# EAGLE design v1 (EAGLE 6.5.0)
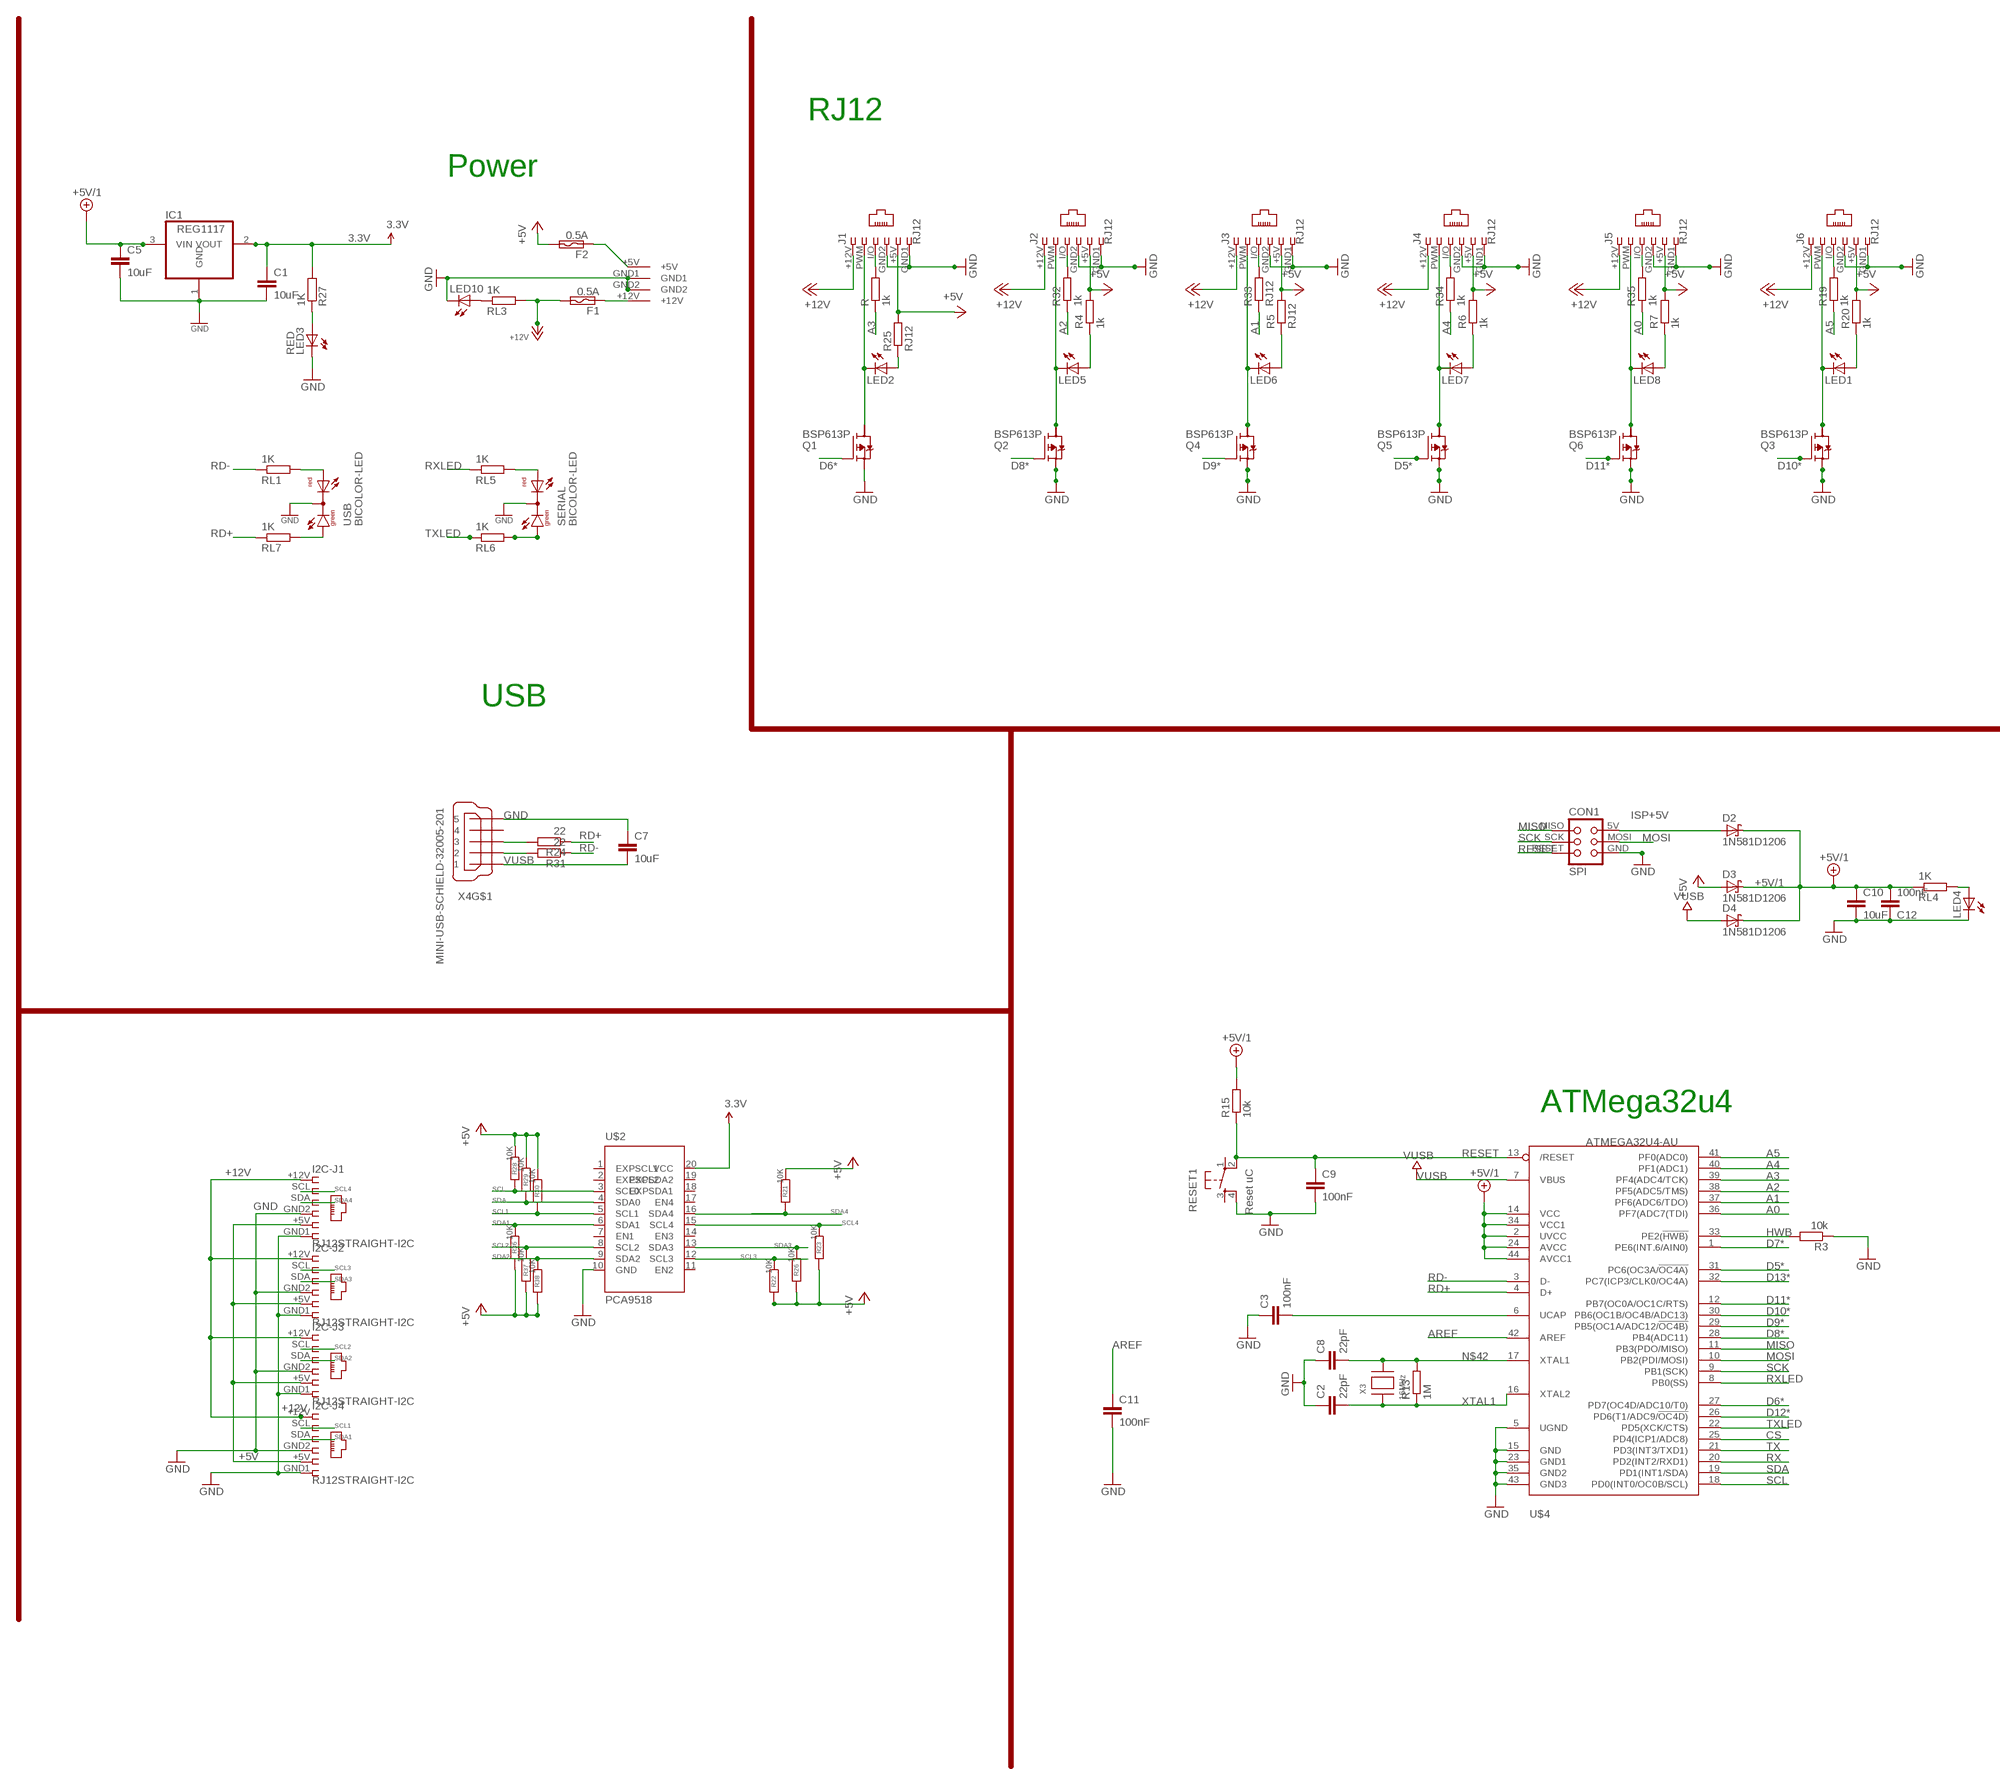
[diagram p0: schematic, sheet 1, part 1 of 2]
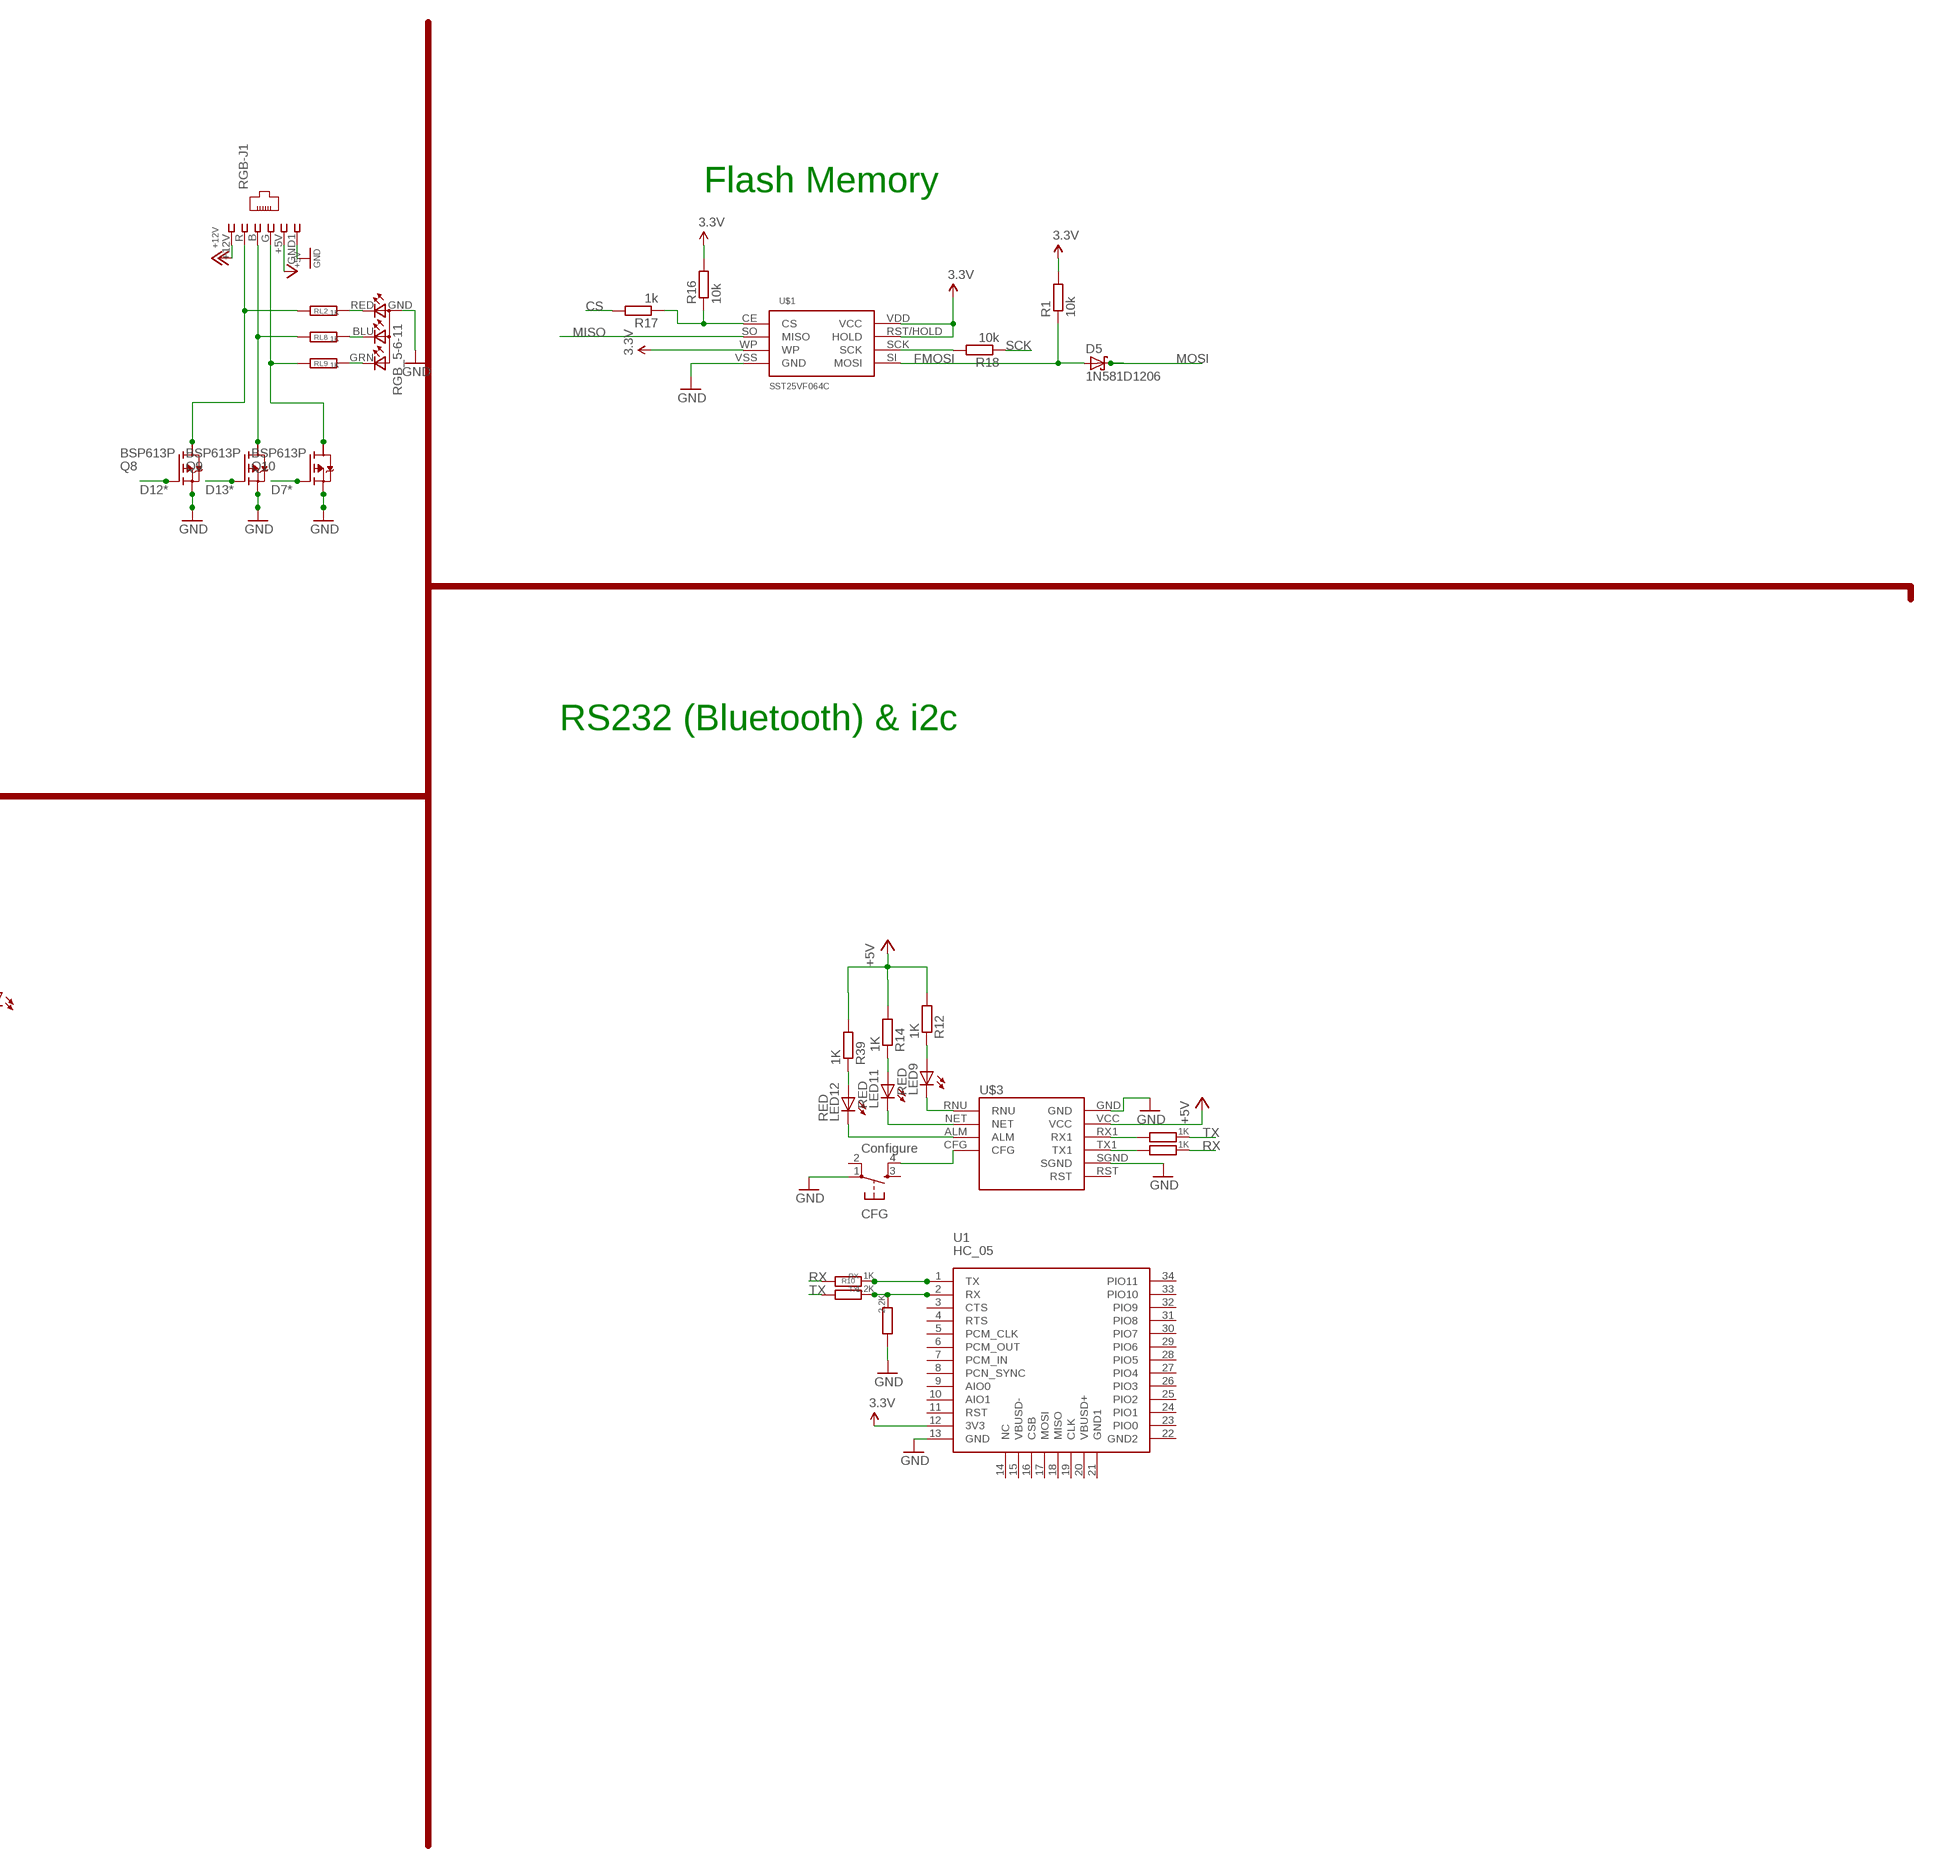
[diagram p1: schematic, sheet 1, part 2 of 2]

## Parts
C1  10uF  C-EUC1206  [C1206]
C2  22pF  C-EUC1206  [C1206]
C3  100nF  C-EUC1206  [C1206]
C5  10uF  C-EUC1206  [C1206]
C7  10uF  C-EUC1206  [C1206]
C8  22pF  C-EUC1206  [C1206]
C9  100nF  C-EUC1206  [C1206]
C10  10uF  C-EUC1206  [C1206]
C11  100nF  C-EUC1206  [C1206]
C12  100nF  C-EUC1206  [C1206]
CFG  Configure  TAC_SWITCHSMD  [TACTILE_SWITCH_SMD]
CON1  SPI  TINYISPT  [TC2030-MCP-NL]
D2  1N581D1206  [LED-1206]
D3  1N581D1206  [LED-1206]
D4  1N581D1206  [LED-1206]
D5  1N581D1206  [LED-1206]
F1  0.5A  POLYSWITCHSMD1812  [C1812]
F2  0.5A  POLYSWITCHSMD1812  [C1812]
I2C-J1  RJ12STRAIGHT-I2C  [RJ12-STRAIGHT-I2C]
I2C-J2  RJ12STRAIGHT-I2C  [RJ12-STRAIGHT-I2C]
I2C-J3  RJ12STRAIGHT-I2C  [RJ12-STRAIGHT-I2C]
I2C-J4  RJ12STRAIGHT-I2C  [RJ12-STRAIGHT-I2C]
IC1  REG1117  [SOT223]
J1  RJ12  RJ12STRAIGHT  [RJ12-STRAIGHT]
J2  RJ12  RJ12STRAIGHT  [RJ12-STRAIGHT]
J3  RJ12  RJ12STRAIGHT  [RJ12-STRAIGHT]
J4  RJ12  RJ12STRAIGHT  [RJ12-STRAIGHT]
J5  RJ12  RJ12STRAIGHT  [RJ12-STRAIGHT]
J6  RJ12  RJ12STRAIGHT  [RJ12-STRAIGHT]
LED1  Blue  LED3MM  [LED3MM]
LED2  Blue  LED3MM  [LED3MM]
LED3  RED  LEDCHIP-LED0805  [CHIP-LED0805]
LED4  RED  LED3MM  [LED3MM]
LED5  Blue  LED3MM  [LED3MM]
LED6  Blue  LED3MM  [LED3MM]
LED7  BLue  LED3MM  [LED3MM]
LED8  Blue  LED3MM  [LED3MM]
LED9  RED  LEDCHIP-LED0805  [CHIP-LED0805]
LED10  RED  LED3MM  [LED3MM]
LED11  RED  LEDCHIP-LED0805  [CHIP-LED0805]
LED12  RED  LEDCHIP-LED0805  [CHIP-LED0805]
Q1  BSP613P  [PG-SOT-223]
Q2  BSP613P  [PG-SOT-223]
Q3  BSP613P  [PG-SOT-223]
Q4  BSP613P  [PG-SOT-223]
Q5  BSP613P  [PG-SOT-223]
Q6  BSP613P  [PG-SOT-223]
Q8  BSP613P  [PG-SOT-223]
Q9  BSP613P  [PG-SOT-223]
Q10  BSP613P  [PG-SOT-223]
R  1k  R-EU_R0805  [R0805]
R1  10k  R-EU_R1206  [R1206]
R2  2.2K  R-EU_R0805  [R0805]
R3  10k  R-EU_M0805  [M0805]
R4  1k  R-EU_R0805  [R0805]
R5  RJ12  R-EU_R0805  [R0805]
R6  1k  R-EU_R0805  [R0805]
R7  1k  R-EU_R0805  [R0805]
R8  1K  R-EU_R0805  [R0805]
R9  1.2K  R-EU_R0805  [R0805]
R10  1K  R-EU_R0805  [R0805]
R11  1K  R-EU_R0805  [R0805]
R12  1K  R-EU_R0805  [R0805]
R13  1M  R-EU_R1206  [R1206]
R14  1K  R-EU_R0805  [R0805]
R15  10k  R-EU_M0805  [M0805]
R16  10k  R-EU_R1206  [R1206]
R17  1k  R-EU_R0805  [R0805]
R18  10k  R-EU_R1206  [R1206]
R19  1k  R-EU_R0805  [R0805]
R20  1k  R-EU_R0805  [R0805]
R21  10K  R-EU_M0805  [M0805]
R22  10K  R-EU_M0805  [M0805]
R23  10K  R-EU_M0805  [M0805]
R24  22  R-EU_M1206  [M1206]
R25  RJ12  R-EU_R0805  [R0805]
R26  10K  R-EU_M0805  [M0805]
R27  1K  R-EU_R0805  [R0805]
R28  10K  R-EU_M0805  [M0805]
R29  10K  R-EU_M0805  [M0805]
R30  10K  R-EU_M0805  [M0805]
R31  22  R-EU_M1206  [M1206]
R32  1k  R-EU_R0805  [R0805]
R33  RJ12  R-EU_R0805  [R0805]
R34  1k  R-EU_R0805  [R0805]
R35  1k  R-EU_R0805  [R0805]
R36  10K  R-EU_M0805  [M0805]
R37  10K  R-EU_M0805  [M0805]
R38  10K  R-EU_M0805  [M0805]
R39  1K  R-EU_R0805  [R0805]
RESET1  Reset uC  TAC_SWITCHSMD  [TACTILE_SWITCH_SMD]
RGB-J1  RJ12  RJ12STRAIGHT-RGB  [RJ12-STRAIGHT-RGB]
RGB_5-6-11  TOPLED-3  [LED-TRICOLOR-THROUGHHOLE]
RL1  1K  R-EU_R0805  [R0805]
RL2  1K  R-EU_M0805  [M0805]
RL3  1K  R-EU_R0805  [R0805]
RL4  1K  R-EU_R0805  [R0805]
RL5  1K  R-EU_R0805  [R0805]
RL6  1K  R-EU_R0805  [R0805]
RL7  1K  R-EU_R0805  [R0805]
RL8  1K  R-EU_M0805  [M0805]
RL9  1K  R-EU_M0805  [M0805]
SERIAL  BICOLOR-LED  [BICOLOR-3MM]
U1  HC_05  [BLUETOOTH_SMD]
U$1  SST25VF064C  [SOIC_8-LEAD]
U$2  PCA9518  [SO20W]
U$3  SZ05-ZIGBEE  [SZ05-ZIGBEE]
U$4  ATMEGA32U4-AU  [TQFP44]
U$6  KPJX-4S-S  [KPJX-4S-S]
USB  BICOLOR-LED  [BICOLOR-3MM]
X3  16MHz  XTALNX6035  [NX6035]
X4  MINI-USB-SCHIELD-32005-201  [32005-201]

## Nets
3.3V [power]: C1.1 IC1.2(VOUT) R1.2 R16.2 R27.2 U1.12(3V3) U$1.RST/HOLD(HOLD) U$1.VDD(VCC) U$1.WP U$2.20(VCC)
+5V [power]: D3.A F2.2 I2C-J1.+5V I2C-J2.+5V I2C-J3.+5V I2C-J4.+5V J1.+5V J2.+5V J3.+5V J4.+5V J5.+5V J6.+5V R4.2 R5.2 R6.2 R7.2 R12.2 R14.2 R20.2 R21.1 R22.2 R23.2 R25.2 R26.2 R28.1 R29.1 R30.1 R36.2 R37.2 R38.2 R39.2 RGB-J1.+5V U$3.VCC
+5V/1 [fine]: C5.1 C10.1 C12.2 D2.C D3.C D4.C IC1.3(VIN) R15.2 RL4.1 U$4.2(UVCC) U$4.14(VCC) U$4.24(AVCC) U$4.34(VCC1) U$4.44(AVCC1)
+12V [power]: F1.2 I2C-J1.+12V I2C-J2.+12V I2C-J3.+12V I2C-J4.+12V J1.+12V J2.+12V J3.+12V J4.+12V J5.+12V J6.+12V RGB-J1.+12V RL3.2
A0: R35.1 U$4.36(PF7(ADC7(TDI))
A1: R33.1 U$4.37(PF6(ADC6/TDO))
A2: R32.1 U$4.38(PF5(ADC5/TMS))
A3: R.1 U$4.39(PF4(ADC4/TCK))
A4: R34.1 U$4.40(PF1(ADC1))
A5: R19.1 U$4.41(PF0(ADC0))
AREF: C11.1 U$4.42(AREF)
CS: R17.2 U$4.25(PD4(ICP1/ADC8))
D2B5: R2.1 R9.1 U1.2(RX)
D5*: Q5.1(G) U$4.31(PC6(OC3A/!OC4A))
D6*: Q1.1(G) U$4.27(PD7(OC4D/ADC10/T0))
D7*: Q10.1(G) U$4.1(PE6(INT.6/AIN0))
D8*: Q2.1(G) U$4.28(PB4(ADC11))
D9*: Q4.1(G) U$4.29(PB5(OC1A/ADC12/!OC4B))
D10*: Q3.1(G) U$4.30(PB6(OC1B/OC4B/ADC13))
D11*: Q6.1(G) U$4.12(PB7(OC0A/OC1C/RTS))
D12*: Q8.1(G) U$4.26(PD6(T1/ADC9/!OC4D))
D13*: Q9.1(G) U$4.32(PC7(ICP3/CLK0/OC4A))
D+USB: R24.2 X4.3
D-USB: R31.2 X4.2
FMOSI: D5.A R1.1 U$1.SI(MOSI)
GND [power]: C1.2 C2.1 C3.1 C5.2 C7.1 C8.1 C9.2 C10.2 C11.2 C12.1 CFG.1 CON1.GND I2C-J1.GND1 I2C-J1.GND2 I2C-J2.GND1 I2C-J2.GND2 I2C-J3.GND1 I2C-J3.GND2 I2C-J4.GND1 I2C-J4.GND2 IC1.1(GND) J1.GND1 J1.GND2 J2.GND1 J2.GND2 J3.GND1 J3.GND2 J4.GND1 J4.GND2 J5.GND1 J5.GND2 J6.GND1 J6.GND2 LED3.C LED4.K(C) LED10.K(C) Q1.3(S) Q2.3(S) Q3.3(S) Q4.3(S) Q5.3(S) Q6.3(S) Q8.3(S) Q9.3(S) Q10.3(S) R2.2 R3.1 RESET1.4 RGB-J1.GND1 RGB_5-6-11.GND(A2) SERIAL.2(C) U1.13(GND) U$1.VSS(GND) U$2.10(GND) U$3.GND U$3.SGND U$4.5(UGND) U$4.15(GND) U$4.23(GND1) U$4.35(GND2) U$4.43(GND3) U$6.GND1 U$6.GND2 USB.2(C) X4.5
GND1 [VIN]: LED9.C U$3.RNU
GND2 [VIN]: LED11.C U$3.NET
GND3 [VIN]: LED12.C U$3.ALM
HWB: R3.2 U$4.33(PE2(!HWB))
ISP+5V: CON1.5V(VCC) D2.A
MISO: CON1.MISO U$1.SO(MISO) U$4.11(PB3(PDO/MISO))
MOSI: CON1.MOSI D5.C U$4.10(PB2(PDI/MOSI))
N$1: J3.PWM LED6.K(C) Q4.2(D)
N$2: J2.I/O R32.2
N$3: J6.I/O R19.2
N$4: LED5.A R4.1
N$5: J4.PWM LED7.K(C) Q5.2(D)
N$6 [aref]: Q10.2(D) RGB-J1.G RL9.1
N$7: J3.I/O R33.2
N$8: RL1.2 USB.3(AR)
N$9: LED1.A R20.1
N$10: R16.1 R17.1 U$1.CE(CS)
N$11: R11.2 U$3.RX1
N$12: LED4.A RL4.2
N$13: RL5.2 SERIAL.3(AR)
N$14: RL7.2 USB.1(AG)
N$15: RL6.2 SERIAL.1(AG)
N$16: C3.2 U$4.6(UCAP)
N$17: LED2.A R25.1
N$18: J1.I/O R.2
N$19: J5.PWM LED8.K(C) Q6.2(D)
N$20: LED3.A R27.1
N$21: J6.PWM LED1.K(C) Q3.2(D)
N$22: LED6.A R5.1
N$23: R18.2 U$1.SCK
N$24: R8.2 U$3.TX1
N$25: LED9.A R12.1
N$26: LED11.A R14.1
N$27: LED12.A R39.1
N$28: J2.PWM LED5.K(C) Q2.2(D)
N$29: J4.I/O R34.2
N$30: LED7.A R6.1
N$32: J5.I/O R35.2
N$33: LED8.A R7.1
N$34: J1.PWM LED2.K(C) Q1.2(D)
N$35: CFG.4 U$3.CFG
N$36: RGB_5-6-11.RED(CRED) RL2.2
N$37: RGB_5-6-11.BLU(CBLUE) RL8.2
N$38: F2.1 U$6.+5V
N$39: F1.1 U$6.+12V
N$40: RGB_5-6-11.GRN(CGREEN) RL9.2
N$42: C8.2 R13.2 U$4.17(XTAL1) X3.P$2
N$50 [aref]: Q9.2(D) RGB-J1.B RL8.1
N$68 [aref]: Q8.2(D) RGB-J1.R RL2.1
N$70: R10.1 U1.1(TX)
N$75: LED10.A RL3.1
RD+: R24.1 RL7.1 U$4.4(D+)
RD-: R31.1 RL1.1 U$4.3(D-)
RESET: C9.1 CON1.RESET R15.1 RESET1.2 U$4.13(/RESET)
RX: R8.1 R10.2 U$4.20(PD2(INT2/RXD1))
RXLED: RL5.1 U$4.8(PB0(SS))
SCK: CON1.SCK R18.1 U$4.9(PB1(SCK))
SCL: R28.2 U$2.3(SCL0) U$4.18(PD0(INT0/OC0B/SCL))
SCL1: I2C-J4.SCL R30.2 U$2.5(SCL1)
SCL2: I2C-J3.SCL R37.1 U$2.8(SCL2)
SCL3: I2C-J2.SCL R22.1 U$2.12(SCL3)
SCL4: I2C-J1.SCL R23.1 U$2.15(SCL4)
SDA: R29.2 U$2.4(SDA0) U$4.19(PD1(INT1/SDA))
SDA1: I2C-J4.SDA R36.1 U$2.6(SDA1)
SDA2: I2C-J3.SDA R38.1 U$2.9(SDA2)
SDA3: I2C-J2.SDA R26.1 U$2.13(SDA3)
SDA4: I2C-J1.SDA R21.2 U$2.16(SDA4)
TX: R9.2 R11.1 U$4.21(PD3(INT3/TXD1))
TXLED: RL6.1 U$4.22(PD5(XCK/CTS))
VUSB: C7.2 D4.A U$4.7(VBUS) X4.1
XTAL1: C2.2 R13.1 U$4.16(XTAL2) X3.P$1
Unconnected: CFG.2 CFG.3 Q1.4(D) Q2.4(D) Q3.4(D) Q4.4(D) Q5.4(D) Q6.4(D) Q8.4(D) Q9.4(D) Q10.4(D) RESET1.1 RESET1.3 U1.3(CTS) U1.4(RTS) U1.5(PCM_CLK) U1.6(PCM_OUT) U1.7(PCM_IN) U1.8(PCN_SYNC) U1.9(AIO0) U1.10(AIO1) U1.11(RST) U1.14(NC) U1.15(VBUSD-) U1.16(CSB) U1.17(MOSI) U1.18(MISO) U1.19(CLK) U1.20(VBUSD+) U1.21(GND1) U1.22(GND2) U1.23(PIO0) U1.24(PIO1) U1.25(PIO2) U1.26(PIO3) U1.27(PIO4) U1.28(PIO5) U1.29(PIO6) U1.30(PIO7) U1.31(PIO8) U1.32(PIO9) U1.33(PIO10) U1.34(PIO11) U$2.1(EXPSCL1) U$2.2(EXPSCL2) U$2.7(EN1) U$2.11(EN2) U$2.14(EN3) U$2.17(EN4) U$2.18(EXPSDA1) U$2.19(EXPSDA2) U$3.RST X4.4 X4.M1(S:S1) X4.M2(S:S2) X4.M3(S:S3) X4.M4(S:S4)

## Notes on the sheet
- RJ12
- Power
- Flash Memory
- RS232 (Bluetooth) & i2c
- USB
- ATMega32u4

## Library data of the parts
C1-C3 C5 C7-C12 = rcl:C-EU: CAPACITOR, European symbol
CFG RESET1 = lpatiny:TAC_SWITCH: Momentary Switch Button commonly used for reset or general input. Spark Fun Electronics SKU : COM-00097
CON1 = lpatiny:TINYISP: CONNECTOR
D2-D5 = lpatiny:1N581*: 1.0A SCHOTTKY BARRIER RECTIFIER
F1 F2 = lpatiny:POLYSWITCH: PolySwitch (TM) Resettable Device
I2C-J1-I2C-J4 J1-J6 RGB-J1 = lpatiny:RJ12: CORCOM Modular RJ Jacks No Shield Source: www.tycoelectronics.com .. ENG_DS_1654001_1099_RJ_L_0507.pdf
IC1 = burr-brown:REG1117: 800mA and 1A Low Dropout (LDO) Positive Regulator 1.8V, 2.5V, 2.85V, 3.3V, 5V, and Adj; MPN: REG1117; OC_FARNELL: 1097566; OC_NEWARK: 14P6981
LED1 LED2 LED4-LED8 LED10 = lpatiny:LED3MM
LED3 LED9 LED11 LED12 = adafruit:LED: LED
Q1-Q6 Q8-Q10 = infineon:BSP613P: SIPMOS (R) Small-Signal-Transistor P-Channel (2 Drain) Source: http://www.infineon.com/dgdl/BSP613P_Rev2.4.pdf; OC_FARNELL: unknown; OC_NEWARK: unknown
R R1 R2 R4-R14 R16-R20 R25 R27 R32-R35 R39 RL1 RL3 RL5-RL7 = rcl:R-EU_: RESISTOR, European symbol
R3 R15 R21-R24 R26 R28-R31 R36-R38 RL2 RL4 RL8 RL9 = resistor:R-EU_: RESISTOR, European symbol
RGB_5-6-11 = lpatiny:TOPLED-3: OSRAM - Hyper Multi TOPLED® (RGB) LB E673, LV E673, LT E673 - Power TOPLED® Enhanced optical Power LED (HOP2000) LS E67B, LA E67B, LO E67B, LY E67B - Hyper Multi TOPLED® Enhanced optical Power LED (HOP2000 / ATON®) LATB T66B - Hyper Multi TOPLED® Hyper-Bright LED LATB T686 Source: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
SERIAL USB = lpatiny:BICOLOR-LED: T-1(3mm) BI-COLOR INDICATOR LAMP Source: Kingbright .. 2_colour_led_.pdf
U1 = Bluetooth HC-05:HC_05: HC-05 Bluetooth Module
U$1 = BertaLib:SST25VF064C
U$2 = lpatiny:PCA9518
U$3 = lpatiny:SZ05-ZIGBEE
U$4 = adafruit:ATMEGA32U4: http://www.ladyada.net/library/eagle
U$6 = lpatiny:KPJX-4S-S
X3 = lpatiny:XTAL: Low cost SMT crystals, no capacitors included
X4 = con-cypressindustries:MINI-USB-SCHIELD-: MINI USB-B Conector Source: www.cypressindustries.com; OC_FARNELL: unknown; OC_NEWARK: unknown

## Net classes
0 default: width 0.305 mm
1 power: width 0.457 mm
2 VIN: width 0.457 mm
3 fine: width 0.305 mm
4 aref: width 0.305 mm

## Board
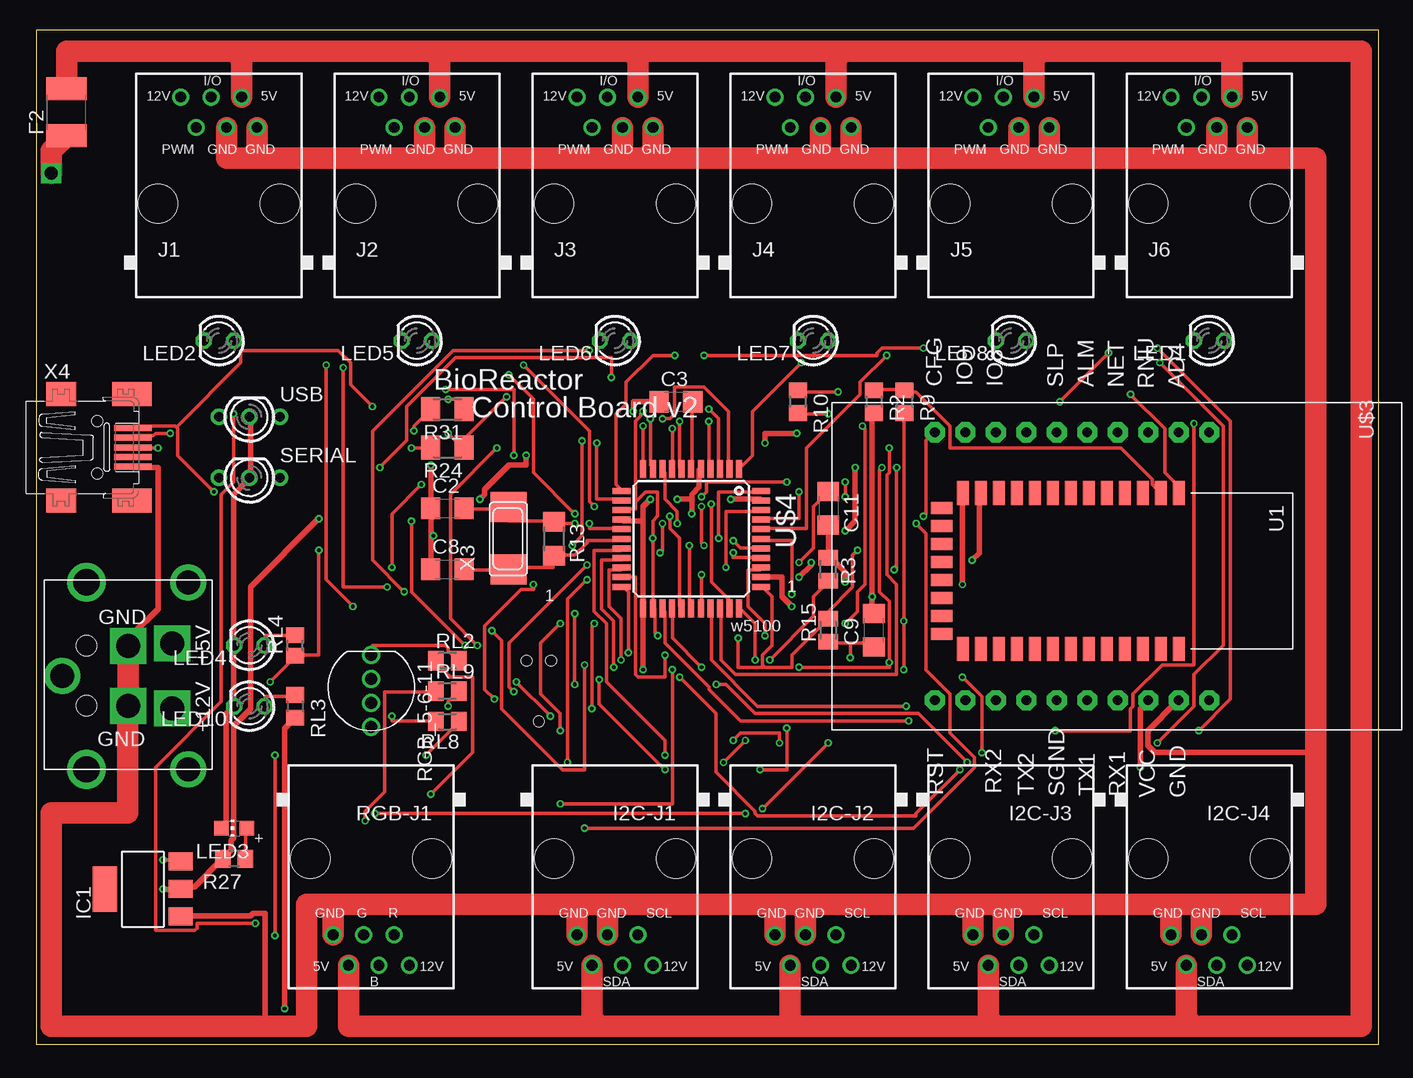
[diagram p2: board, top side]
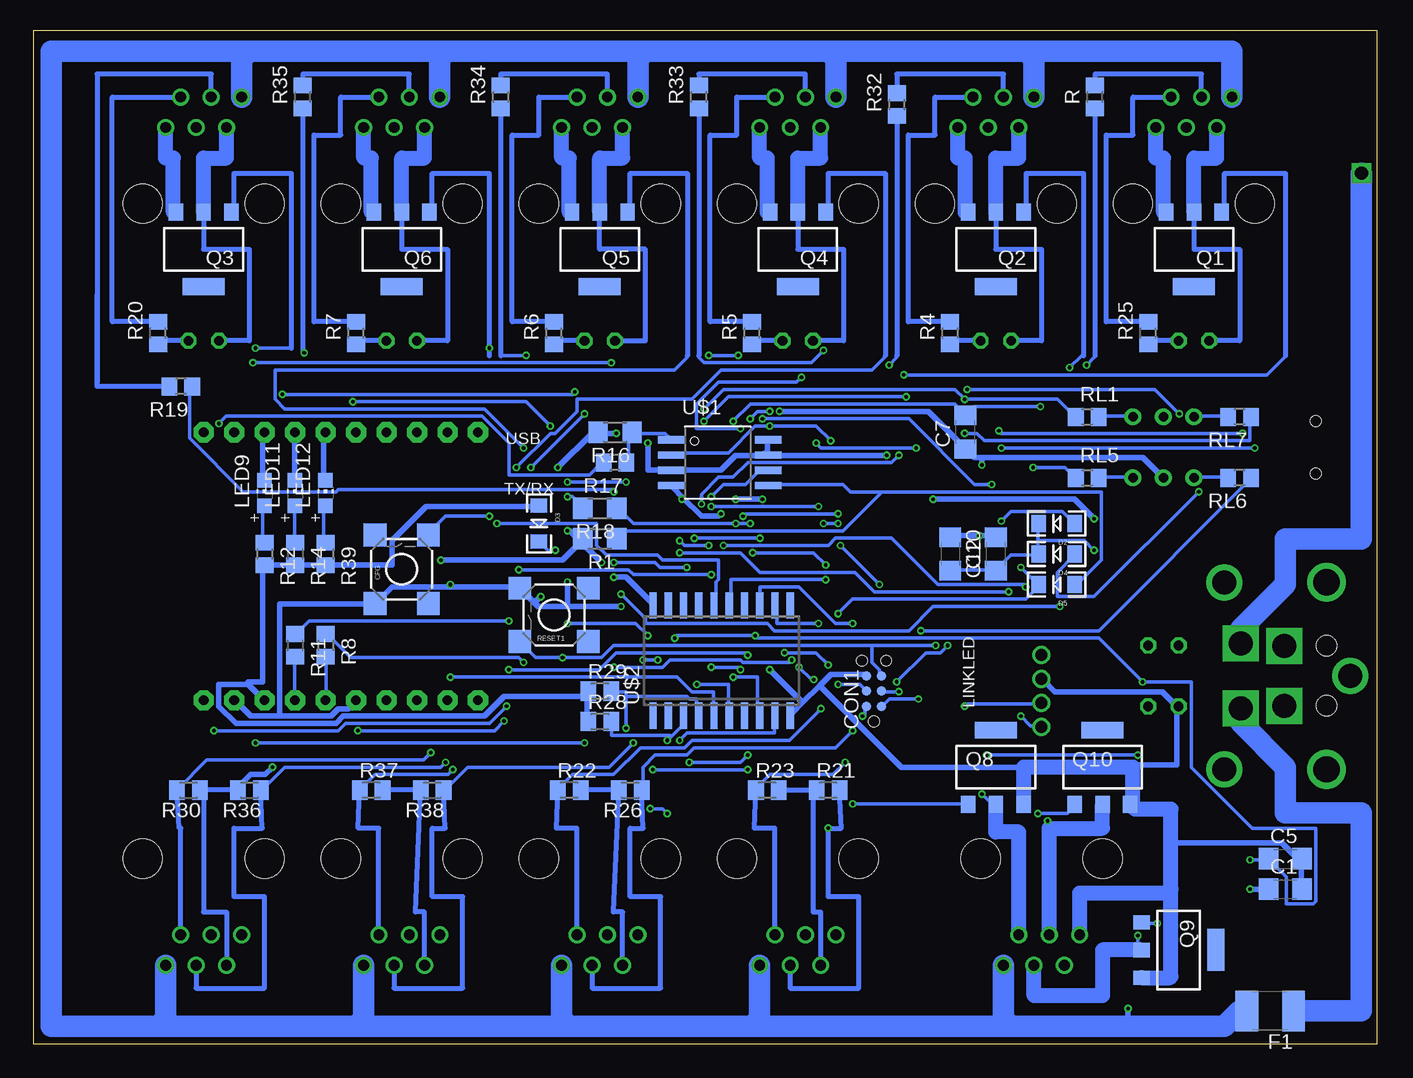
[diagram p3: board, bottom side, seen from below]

Size 111.94 x 84.57 mm. Coordinates in mm from the lower left corner, seen from the top.
Outline: 0,0 111.94,0 111.94,84.57 0,84.57 0,0
Copper layers (1*16): Top 0.035mm / dielectric 1.5mm / Bottom 0.035mm
Design rules "Fusion_eagle_rule_v1.1": minimum track width 6mil, minimum drill 12mil, track to track 6mil, track to pad 6mil, pad to pad 6mil, via to via 6mil, smd to smd 0mil, copper to edge 10mil, drill to drill 10mil, minimum pad ring 10mil, minimum via ring 6mil, stop-mask expansion 2mil, vias tented up to drill 100mil, thermal gap 10mil
bKeepout: area -1.3,57.4 to 114.3,85.3; area -7.6,54.9 to 108,82.8
tRestrict: area -6.3,58.7 to 116.8,85.3; area 22.9,-4.8 to 118.1,16.8
bRestrict: area -6.3,58.7 to 116.8,85.3; area 22.9,-4.8 to 118.1,16.8
vRestrict: area 47,34.5 to 62.2,38.4; area 47,35.8 to 50.8,49.8; area 58.4,37.1 to 62.2,49.8; area 47,46 to 62.2,49.8; area 47,25.7 to 62.2,29.5

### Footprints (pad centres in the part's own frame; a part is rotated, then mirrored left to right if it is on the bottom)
C1206 = smd 1.6 x 1.8: 1 -1.4,0; 2 1.4,0
TACTILE_SWITCH_SMD = smd 1.905 x 1.905: 1 -2.857,2.223; 2 2.857,2.223; 3 -2.857,-2.223; 4 2.857,-2.223
TC2030-MCP-NL = smd 0.787 x 0.787: 5V 1.27,0.635; GND 3.81,0.635; MISO 1.27,-0.635; MOSI 2.54,0.635; RESET 3.81,-0.635; SCK 2.54,-0.635 | hole 0.889: 0,0; 5.08,-1.016; 5.08,1.016
LED-1206 = smd 1.2 x 1.4: A -1.5,0; C 1.5,0
C1812 = smd 1.9 x 3.4: 1 -1.95,0; 2 1.95,0
RJ12-STRAIGHT-I2C = drill 0.9 pad 1.4: +5V 1.905,8.89; +12V -3.175,8.89; GND1 3.175,6.35; GND2 0.635,6.35; SCL -1.905,6.35; SDA -0.635,8.89 | hole 3.251: -5.08,0; 5.08,0
SOT223 = smd 1.499 x 2.007: 1 -2.261,-3.15; 2 0.025,-3.15; 3 2.311,-3.15 | smd 3.81 x 2.007: 4 0,3.15
RJ12-STRAIGHT = drill 0.9 pad 1.4: +5V 1.905,8.89; +12V -3.175,8.89; GND1 3.175,6.35; GND2 0.635,6.35; I/O -0.635,8.89; PWM -1.905,6.35 | hole 3.251: -5.08,0; 5.08,0
LED3MM = drill 0.813 octagon: A -1.27,0; K 1.27,0
CHIP-LED0805 = smd 1.2 x 1.2: A 0,-1.05; C 0,1.05
PG-SOT-223 = smd 1.2 x 1.4: 1 -2.311,-3.099; 2 0,-3.099; 3 2.311,-3.099 | smd 3.5 x 1.4: 4 0,3.099
R0805 = smd 1.3 x 1.5: 1 -0.95,0; 2 0.95,0
R1206 = smd 1.6 x 1.803: 1 -1.422,0; 2 1.422,0
M0805 = smd 1.3 x 1.6: 1 -0.95,0; 2 0.95,0
M1206 = smd 1.6 x 2: 1 -1.4,0; 2 1.4,0
RJ12-STRAIGHT-RGB = drill 0.9 pad 1.4: +5V 1.905,8.89; +12V -3.175,8.89; B -0.635,8.89; G 0.635,6.35; GND1 3.175,6.35; R -1.905,6.35 | hole 3.251: -5.08,0; 5.08,0
LED-TRICOLOR-THROUGHHOLE = drill 1: BLU 3,0; GND -1,0; GRN 1,0; RED -3,0
R0805' = smd 1.3 x 1.5: 1 -0.85,0; 2 0.85,0
BICOLOR-3MM = drill 0.8 pad 1.4: 1 -2.54,0; 2 0,0; 3 2.54,0
BLUETOOTH_SMD = smd 2 x 1: 1 -6.35,3.81; 2 -6.35,2.31; 3 -6.35,0.81; 4 -6.35,-0.69; 5 -6.35,-2.19; 6 -6.35,-3.69; 7 -6.35,-5.19; 8 -6.35,-6.69; 9 -6.35,-8.19; 10 -6.35,-9.69; 11 -6.35,-11.19; 12 -6.35,-12.69; 13 -6.35,-14.19; 22 6.65,-14.19; 23 6.65,-12.69; 24 6.65,-11.19; 25 6.65,-9.69; 26 6.65,-8.19; 27 6.65,-6.69; 28 6.65,-5.19; 29 6.65,-3.69; 30 6.65,-2.19; 31 6.65,-0.69; 32 6.65,0.81; 33 6.65,2.31; 34 6.65,3.81 | smd 1 x 1.8: 14 -5.1,-15.94; 15 -3.6,-15.94; 16 -2.1,-15.94; 17 -0.6,-15.94; 18 0.9,-15.94; 19 2.4,-15.94; 20 3.9,-15.94; 21 5.4,-15.94
SOIC_8-LEAD = smd 0.61 x 2.21: CE -1.905,-2.934; RST/HOLD -0.635,5.156; SCK 0.635,5.156; SI 1.905,5.156; SO -0.635,-2.934; VDD -1.905,5.156; VSS 1.905,-2.934; WP 0.635,-2.934
SO20W = smd 0.6 x 2.2: 1 -5.715,-4.6; 2 -4.445,-4.6; 3 -3.175,-4.6; 4 -1.905,-4.6; 5 -0.635,-4.6; 6 0.635,-4.6; 7 1.905,-4.6; 8 3.175,-4.6; 9 4.445,-4.6; 10 5.715,-4.6; 11 5.715,4.6; 12 4.445,4.6; 13 3.175,4.6; 14 1.905,4.6; 15 0.635,4.6; 16 -0.635,4.6; 17 -1.905,4.6; 18 -3.175,4.6; 19 -4.445,4.6; 20 -5.715,4.6
SZ05-ZIGBEE = drill 0.8 pad 1.676 octagon: 6 -11.415,13.971; 7 -11.415,11.431; 11 -11.415,1.271; 12 -11.415,-1.269; 13 -11.415,-3.809; 14 -11.415,-6.349; 17 10.925,-6.349; 18 10.925,-3.809; 19 10.925,-1.269; 25 10.925,13.971; ALM -11.415,3.811; CFG -11.415,-8.889; GND 10.925,11.431; NET -11.415,6.351; RNU -11.415,8.891; RST 10.925,-8.889; RX1 10.925,6.351; SGND 10.925,1.271; TX1 10.925,3.811; VCC 10.925,8.891
TQFP44 = smd 1.5 x 0.5: 1 -5.8,4; 2 -5.8,3.2; 3 -5.8,2.4; 4 -5.8,1.6; 5 -5.8,0.8; 6 -5.8,0; 7 -5.8,-0.8; 8 -5.8,-1.6; 9 -5.8,-2.4; 10 -5.8,-3.2; 11 -5.8,-4; 23 5.8,-4; 24 5.8,-3.2; 25 5.8,-2.4; 26 5.8,-1.6; 27 5.8,-0.8; 28 5.8,0; 29 5.8,0.8; 30 5.8,1.6; 31 5.8,2.4; 32 5.8,3.2; 33 5.8,4 | smd 0.5 x 1.5: 12 -4,-5.8; 13 -3.2,-5.8; 14 -2.4,-5.8; 15 -1.6,-5.8; 16 -0.8,-5.8; 17 0,-5.8; 18 0.8,-5.8; 19 1.6,-5.8; 20 2.4,-5.8; 21 3.2,-5.8; 22 4,-5.8; 34 4,5.8; 35 3.2,5.8; 36 2.4,5.8; 37 1.6,5.8; 38 0.8,5.8; 39 0,5.8; 40 -0.8,5.8; 41 -1.6,5.8; 42 -2.4,5.8; 43 -3.2,5.8; 44 -4,5.8
KPJX-4S-S = drill 2 square: +5V 2.7,1.35; +12V -2.7,1.35; GND1 -2.5,5; GND2 2.5,5 | drill 2: P$1 -7.8,0; P$2 7.8,0; P$11 0,10.5 | drill 2.2: P$3 -7.8,8.5; P$4 7.8,8.5 | hole 1.7: -2.5,8.5; 2.5,8.5
NX6035 = smd 2.5 x 3: P$1 2.665,0; P$2 -2.565,0
32005-201 = smd 3.1 x 0.5: 1 3,1.6; 2 3,0.8; 3 3,0; 4 3,-0.8; 5 3,-1.6 | smd 2.5 x 2: M1 -3,-4.45; M2 -3,4.45 | smd 3.3 x 2: M3 2.9,4.45; M4 2.9,-4.45 | hole 0.9: 0,2.2; 0,-2.2

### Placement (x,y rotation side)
C1  7.62,12.95 0 bottom
C2  34.29,44.7 0 top
C3  53.34,53.59 0 top
C5  7.62,15.49 0 bottom
C7  34.29,51.05 90 bottom
C8  34.29,39.62 0 top
C9  69.85,34.54 90 top
C10  31.75,40.89 90 bottom
C11  66.04,44.7 270 top
C12  35.56,40.89 270 bottom
CFG  81.28,39.62 90 bottom
CON1  41.91,26.92 90 bottom
D2  26.67,43.43 180 bottom
D3  69.85,43.43 270 bottom
D4  26.67,40.89 180 bottom
D5  26.67,38.35 180 bottom
F1  8.89,2.79 180 bottom
F2  2.54,77.72 90 top
I2C-J1  48.26,15.49 180 top
I2C-J2  64.77,15.49 180 top
I2C-J3  81.28,15.49 180 top
I2C-J4  97.79,15.49 180 top
IC1  8.89,12.95 90 top
J1  15.24,70.1 0 top
J2  31.75,70.1 0 top
J3  48.26,70.1 0 top
J4  64.77,70.1 0 top
J5  81.28,70.1 0 top
J6  97.79,70.1 0 top
LED1  97.79,58.67 180 top
LED2  15.24,58.67 180 top
LED3  16.51,18.03 90 top
LED4  17.78,33.27 180 top
LED5  31.75,58.67 180 top
LED6  48.26,58.67 180 top
LED7  64.77,58.67 180 top
LED8  81.28,58.67 180 top
LED9  92.71,45.97 0 bottom
LED10  17.78,28.19 180 top
LED11  90.17,45.97 0 bottom
LED12  87.63,45.97 0 bottom
Q1  15.24,66.29 180 bottom
Q2  31.75,66.29 180 bottom
Q3  97.79,66.29 180 bottom
Q4  48.26,66.29 180 bottom
Q5  64.77,66.29 180 bottom
Q6  81.28,66.29 180 bottom
Q8  31.75,23.11 0 bottom
Q9  16.51,7.87 270 bottom
Q10  22.86,23.11 0 bottom
R  23.5,78.99 90 bottom
R1  64.77,42.16 180 bottom
R2  69.85,53.59 270 top
R3  66.04,39.62 270 top
R4  35.56,59.31 90 bottom
R5  52.07,59.31 90 bottom
R6  68.58,59.31 90 bottom
R7  85.09,59.31 90 bottom
R8  87.63,33.27 270 bottom
R9  72.39,53.59 270 top
R10  63.5,53.59 270 top
R11  90.17,33.27 270 bottom
R12  92.71,40.89 270 bottom
R13  43.18,42.16 270 top
R14  90.17,40.89 270 bottom
R15  66.04,34.54 90 top
R16  63.5,51.05 180 bottom
R17  63.5,48.51 180 bottom
R18  64.77,44.7 180 bottom
R19  99.69,54.86 180 bottom
R20  101.6,59.31 90 bottom
R21  45.72,21.21 0 bottom
R22  67.31,21.21 0 bottom
R23  50.8,21.21 0 bottom
R24  34.29,49.78 180 top
R25  19.05,59.31 90 bottom
R26  62.23,21.21 180 bottom
R27  16.51,15.49 180 top
R28  64.77,26.92 0 bottom
R29  64.77,29.46 0 bottom
R30  99.06,21.21 180 bottom
R31  34.29,52.96 180 top
R32  40.01,78.36 90 bottom
R33  56.52,78.99 90 bottom
R34  73.03,78.99 90 bottom
R35  89.53,78.99 90 bottom
R36  93.98,21.21 180 bottom
R37  83.82,21.21 0 bottom
R38  78.74,21.21 180 bottom
R39  87.63,40.89 270 bottom
RESET1  68.58,35.81 180 bottom
RGB-J1  27.94,15.49 180 top
RGB_5-6-11  27.94,29.46 270 top
RL1  24.13,52.32 0 bottom
RL2  34.29,32 0 top
RL3  21.59,28.19 270 top
RL4  1K  [R0805']  21.59,33.27 90 top
RL5  24.13,47.24 0 bottom
RL6  11.43,47.24 180 bottom
RL7  11.43,52.32 180 bottom
RL8  34.29,26.92 180 top
RL9  34.29,29.46 0 top
SERIAL  17.78,47.24 0 top
U1  91.44,39.62 270 top
U$1  55.88,48.51 270 bottom
U$2  54.61,32 0 bottom
U$3  83.82,39.62 270 top
U$4  54.61,42.16 270 top
U$6  12.7,30.73 90 top
USB  17.78,52.32 0 top
X3  39.37,42.16 90 top
X4  5.08,49.78 0 top

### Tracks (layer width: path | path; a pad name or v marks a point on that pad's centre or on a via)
3.3V  (via drill 0.3)
  Top 0.457: v78.03,40.39 78.64,41 78.64,45.87 U1.12 | v63.6,38.96 64.62,39.98 v64.62,40.18 | v10.57,12.95 11.99,12.95 IC1.2 12.19,13.16 13.21,13.16 15.44,15.39 R27.2 15.65,15.6 16.26,16.2 16.26,17.02 16.46,17.22 16.46,26.57 17.88,27.99 17.88,38.15 v23.57,43.84 | v63.4,50.95 60.76,50.95 v60.76,50.14 | v36.98,45.47 37.39,45.87 37.39,46.28 39.42,48.31 40.84,48.31 v40.84,49.12 | v67.46,42.82 68.28,43.64 v68.28,48.11
  Bottom 0.457: v78.03,40.39 67.87,40.39 66.24,42.01 R1.2 | v63.6,38.96 62.59,38.96 60.35,36.73 U$2.20 | v64.62,40.18 66.24,41.81 R1.2 | v10.57,12.95 9.14,12.95 C1.1 | U$1.RST/HOLD 50.8,49.33 50.8,50.34 U$1.VDD | v63.4,50.95 64.82,50.95 R16.2 65.02,50.95 65.43,50.95 v68.28,48.11 | v60.76,50.14 60.76,47.9 58.93,47.9 U$1.WP 58.73,47.9 54.66,47.9 53.44,49.12 51.21,49.12 51,49.33 U$1.RST/HOLD | v23.57,43.84 25.2,45.47 v36.98,45.47 | v40.84,49.12 50.6,49.12 U$1.RST/HOLD | v67.46,42.82 67.26,42.82 66.45,42.01 R1.2
+5V  (via drill 0.3)
  Top 0.457: v92.05,23.11 92.05,27.99 92.66,28.6 U$3.VCC
  Top 1.778: F2.2 2.54,82.8 16.51,82.8 | 16.51,82.8 33.02,82.8 | 33.02,82.8 49.53,82.8 | 49.53,82.8 67.31,82.8 | 67.31,82.8 83.82,82.8 | 83.82,82.8 100.33,82.8 | 100.33,82.8 110.49,82.8 110.49,1.52 96.52,1.52 | 96.52,1.52 80.01,1.52 | 80.01,1.52 63.5,1.52 | 63.5,1.52 46.99,1.52 | 46.99,1.52 26.04,1.52 RGB-J1.+5V | J1.+5V 17.14,82.17 16.51,82.8 | J2.+5V 33.66,82.17 33.02,82.8 | J3.+5V 50.16,82.17 49.53,82.8 | J4.+5V 66.67,82.17 67.31,82.8 | J5.+5V 83.19,82.17 83.82,82.8 | J6.+5V 99.69,82.17 100.33,82.8 | I2C-J1.+5V 46.35,2.16 46.99,1.52 | I2C-J2.+5V 62.87,2.16 63.5,1.52 | I2C-J3.+5V 79.38,2.16 80.01,1.52 | I2C-J4.+5V 95.89,2.16 96.52,1.52
  Bottom 0.406: I2C-J2.+5V 62.87,11.05 63.63,11.05 R26.2 R22.2 66.04,21.21 66.04,21.84 | I2C-J3.+5V 79.38,11.05 80.14,11.05 R38.2 R37.2 | I2C-J4.+5V 95.89,11.05 97.79,11.05 97.79,21.21 R30.1 R36.2 | R21.1 46.99,21.21 | 46.99,21.21 46.99,20.57 | 46.99,20.57 46.99,11.05 46.35,11.05 I2C-J1.+5V | R23.2 46.99,21.21 | 46.99,21.21 46.99,20.57 | R25.2 22.54,60.26 22.54,75.82 20.32,75.82 20.32,78.99 J1.+5V | R4.2 39.05,60.26 39.05,75.82 36.83,75.82 36.83,78.99 J2.+5V | R5.2 55.56,60.26 55.56,75.82 53.34,75.82 53.34,78.99 J3.+5V | R6.2 72.07,60.26 72.07,75.82 69.85,75.82 69.85,78.99 J4.+5V | R7.2 88.58,60.26 88.58,75.82 86.36,75.82 86.36,78.99 J5.+5V | R20.2 105.41,60.26 105.41,78.99 J6.+5V
  Bottom 0.457: D3.A 69.9,44.86 79.25,44.86 82.09,42.01 82.09,39.98 87.58,39.98 R39.2 87.78,39.98 90.02,39.98 R14.2 90.22,39.98 92.66,39.98 R12.2 92.86,39.78 92.86,30.23 94.08,30.23 94.08,30.02 | R28.1 65.84,26.98 65.84,29.41 R29.1 66.04,29.01 72.75,29.01 74.37,27.38 86.16,27.38 86.77,26.77 95.1,26.77 96.52,28.19 96.52,30.02 94.08,30.02 | 94.08,30.02 92.86,28.8 U$3.VCC | v92.05,23.11 92.66,22.5 93.88,22.5 95.1,21.29 R36.2
+5V/1  (via drill 0.3)
  Top 0.305: v68.48,41.2 68.07,40.79 68.07,38.15 66.04,36.12 66.04,35.51 | 66.04,35.51 R15.2 66.04,35.51 | 60.66,31.55 60.76,31.45 62.99,31.45 62.99,32.46 66.04,35.51 | 60.66,31.55 60.55,31.65 60.55,32.46 61.37,33.27 61.37,37.34 60.55,38.15 U$4.34 | 50.09,45.36 50.8,46.08 51.82,46.08 51.82,44.04 51.41,43.64 v51.41,42.21 51.41,36.52 U$4.24 51.61,36.32 51.61,34.29 v51.82,34.09 | 50.09,45.36 49.99,45.26 49.99,44.65 48.97,44.65 U$4.14 | v52.22,52.17 52.83,52.17 53.24,52.58 53.24,54.81 55.68,54.81 57.71,52.78 57.71,48.11 U$4.2 | v50.6,52.78 50.39,52.58 50.39,52.38 49.99,51.97 49.99,45.47 50.09,45.36 | v56.9,42.21 56.9,46.08 60.35,46.08 U$4.44 | v58.52,33.88 58.52,31.45 60.55,31.45 60.66,31.55 | v10.57,15.39 11.99,15.39 IC1.3 | v23.57,41.2 23.57,32.46 21.74,32.46 RL4.1 21.54,32.26 v19.51,30.23
  Bottom 0.305: v68.48,41.2 69.09,41.2 69.7,41.81 D3.C | v52.22,52.17 51.61,52.78 v50.6,52.78 | v51.41,42.21 v56.9,42.21 | v58.52,33.88 58.32,34.09 v51.82,34.09 51.61,33.88 23.16,33.88 v19.51,30.23 15.44,30.23 15.44,23.11 10.36,18.03 5.08,18.03 5.08,11.94 5.28,11.74 7.52,11.74 7.52,13.97 8.94,15.39 C5.1 9.14,15.39 v10.57,15.39 | C12.2 35.56,39.57 31.9,39.57 C10.1 31.7,39.57 30.48,40.79 28.25,40.79 D4.C 28.25,41 28.25,42.01 | 28.25,42.01 28.25,43.43 D2.C | v23.57,41.2 24.38,42.01 28.25,42.01
+12V  (via drill 0.3)
  Top 0.457: v20.73,3 20.73,26.37 21.54,27.18 RL3.2
  Bottom 0.457: v20.73,3 20.73,2.39 20.73,1.52
  Bottom 1.778: F1.2 11.43,2.79 12.7,1.52 20.73,1.52 30.48,1.52 | 30.48,1.52 52.07,1.52 | 52.07,1.52 67.31,1.52 | 67.31,1.52 85.09,1.52 | 85.09,1.52 101.6,1.52 | 101.6,1.52 110.49,1.52 110.49,82.8 93.98,82.8 | 93.98,82.8 77.47,82.8 | 77.47,82.8 60.96,82.8 | 60.96,82.8 45.72,82.8 | 45.72,82.8 29.21,82.8 | 29.21,82.8 12.06,82.8 J1.+12V | J3.+12V 45.09,82.17 45.72,82.8 | J4.+12V 61.59,82.17 60.96,82.8 | J5.+12V 78.11,82.17 77.47,82.8 | J6.+12V 94.61,82.17 93.98,82.8 | J2.+12V 28.57,82.17 29.21,82.8 | I2C-J4.+12V 100.97,2.16 101.6,1.52 | I2C-J3.+12V 84.45,2.16 85.09,1.52 | I2C-J2.+12V 67.94,2.16 67.31,1.52 | I2C-J1.+12V 51.44,2.16 52.07,1.52 | RGB-J1.+12V 31.11,2.16 30.48,1.52
A0  (via drill 0.3)
  Top 0.305: v60.76,34.09 60.76,35.1 59.33,36.52 59.33,39.57 60.35,39.57 U$4.36 | v67.46,35.1 68.48,36.12 68.48,37.74 69.09,38.35 69.09,51.36 v68.89,51.56 | v89.41,57.66 v85.34,53.59
  Bottom 0.305: v60.76,34.09 61.77,35.1 v67.46,35.1 | v68.89,51.56 70.92,53.59 v85.34,53.59 | v89.41,57.66 89.53,57.72
  Bottom 0.406: R35.1 89.53,57.72
A1  (via drill 0.3)
  Top 0.305: v58.12,41 58.12,40.59 60.35,40.59 U$4.37 | v30.68,37.74 28.04,40.39 28.04,51.16 34.75,57.86 v46.13,57.86
  Bottom 0.305: v58.12,41 53.03,41 51.41,39.37 43.48,39.37 41.86,37.74 v30.68,37.74 | v46.13,57.86 47.14,56.84 56.08,56.84 56.49,57.25 56.52,57.4
  Bottom 0.406: R33.1 56.52,57.4
A2  (via drill 0.3)
  Top 0.305: v58.12,42.01 58.73,41.4 60.35,41.4 U$4.38 | v55.68,41.6 55.47,41.81 v55.47,44.86 | v46.53,44.86 46.13,45.26 46.13,51.16 v40.64,56.64
  Bottom 0.305: v58.12,42.01 57.71,41.6 v55.68,41.6 | v46.53,44.86 v55.47,44.86 | v40.64,56.64 40.03,57.25 40.01,57.4
  Bottom 0.406: R32.1 40.01,57.4
A3  (via drill 0.3)
  Top 0.305: v62.99,37.54 62.99,42.01 60.55,42.01 U$4.39 | v26.42,36.52 24.18,38.76 v24.18,56.64
  Bottom 0.305: v62.99,37.54 60.96,35.51 60.96,35.1 50.8,35.1 50.19,34.49 39.01,34.49 36.98,36.52 v26.42,36.52 | v24.18,56.64 23.57,57.25 23.5,57.4
  Bottom 0.406: R.1 23.5,57.4
A4  (via drill 0.3)
  Top 0.305: v70.92,57.45 68.68,55.22 68.68,54.2 64.21,49.73 64.21,43.03 60.55,43.03 U$4.40
  Bottom 0.305: v70.92,57.45 72.95,57.45 73.03,57.45
  Bottom 0.406: R34.1 73.03,57.45 73.03,57.4
A5  (via drill 0.3)
  Top 0.305: v63.6,46.08 63.6,43.84 60.55,43.84 U$4.41
  Bottom 0.305: v63.6,46.08 63.8,46.28 86.56,46.28 86.77,46.08 94.49,46.08 98.96,50.55 98.96,54.81 98.75,54.81 R19.1
AREF  (via drill 0.3)
  Top 0.305: v57.51,39.78 57.51,44.45 60.35,44.45 U$4.42 | v63.6,40.18 64.82,41.4 64.82,44.86 66.04,46.08 C11.1
  Bottom 0.305: v57.51,39.78 59.74,39.78 60.15,40.18 v63.6,40.18
CS  (via drill 0.3)
  Top 0.305: v72.75,26.98 58.73,26.98 56.08,29.62 56.08,29.82 52.43,33.48 52.43,36.12 52.22,36.32 U$4.25 | v84.94,26.16 91.24,26.16 91.24,27.99 91.44,28.19 91.44,29.21 93.88,31.65 96.52,31.65 v96.52,51.76
  Bottom 0.305: v72.75,26.98 73.56,26.16 v84.94,26.16 | v96.52,51.76 95.91,52.38 74.57,52.38 72.34,50.14 72.34,47.5 65.63,47.5 64.62,48.51 R17.2
D2B5
  Top 0.305: R2.1 69.9,54.61 72.34,54.61 R9.1 72.54,54.41 73.36,54.41 76.2,51.56 76.2,49.73 90.42,49.73 93.07,47.09 93.07,46.68 93.67,46.08 U1.2
D5*  (via drill 0.3)
  Top 0.305: v71.12,49.73 71.12,47.7 70.92,47.5 70.92,39.17 71.73,38.35 71.73,30.84 58.32,30.84 57.1,32.05 57.1,36.32 U$4.31
  Bottom 0.305: v71.12,49.73 74.37,52.98 91.03,52.98 91.85,53.8 91.85,56.24 58.52,56.24 57.51,57.25 57.47,57.4
  Bottom 0.406: Q5.1 62.23,69.39 62.23,72.64 57.47,72.64 57.47,57.4
D6*  (via drill 0.3)
  Top 0.305: v52.83,44.04 52.83,43.03 53.65,42.21 53.65,36.52 U$4.27 | v44.91,44.25 41.45,47.7 41.45,53.8 v39.42,55.83
  Bottom 0.305: v52.83,44.04 52.63,44.25 v44.91,44.25 | v39.42,55.83 9.14,55.83 7.72,57.25 7.62,57.4
  Bottom 0.406: Q1.1 12.7,69.39 12.7,72.64 7.62,72.64 7.62,57.4
D7*  (via drill 0.3)
  Top 0.305: v59.13,19.25 v28.25,19.25 | v66.04,25.15 v60.55,19.66 | v93.47,25.15 96.52,28.19 96.52,30.84 98.96,33.27 98.96,51.56 v93.67,56.84 | v63.8,56.84 59.74,52.78 59.74,49.12 58.73,48.11 U$4.1
  Bottom 0.305: v28.25,19.25 25.81,19.25 25.2,19.86 Q10.1 | v59.13,19.25 59.54,19.66 v60.55,19.66 | v93.47,25.15 v66.04,25.15 | v63.8,56.84 v93.67,56.84
D8*  (via drill 0.3)
  Top 0.305: v54.46,41.6 54.46,36.52 U$4.28 | v29.26,38.15 25.6,38.15 v25.6,56.44
  Bottom 0.305: v54.46,41.6 45.72,41.6 45.11,42.21 40.44,42.21 36.58,38.35 29.46,38.35 v29.26,38.15 | v25.6,56.44 24.59,57.45 24.45,57.45
  Bottom 0.406: Q2.1 29.21,69.39 29.21,72.64 24.45,72.64 24.45,57.45 24.45,57.4
D9*  (via drill 0.3)
  Top 0.305: v55.47,39.17 55.47,36.52 U$4.29 | v71.53,39.57 71.73,39.78 v71.73,48.11
  Bottom 0.305: v55.47,39.17 61.98,39.17 62.38,39.57 v71.53,39.57 | v71.73,48.11 68.89,50.95 68.48,50.95 66.65,52.78 66.65,53.8 57.1,53.8 54.66,56.24 42.06,56.24 41.05,57.25 40.96,57.4
  Bottom 0.406: Q4.1 45.72,69.39 45.72,72.64 40.96,72.64 40.96,57.4
D10*  (via drill 0.3)
  Top 0.305: v72.54,28.19 60.15,28.19 56.29,32.05 56.29,36.32 U$4.30 | v96.93,26.16 99.57,28.8 99.57,51.97 v93.47,58.06
  Bottom 0.305: v72.54,28.19 73.97,26.77 85.95,26.77 86.56,26.16 v96.93,26.16 | v93.47,58.06 90.63,58.06 90.49,58.06
  Bottom 0.406: Q3.1 95.25,69.39 95.25,72.64 90.49,72.64 90.49,58.06 90.49,58.04
D11*  (via drill 0.3)
  Top 0.305: v53.24,57.45 51.41,57.45 49.17,55.22 49.17,53.39 48.36,52.58 48.36,46.68 48.77,46.28 U$4.12 | v55.68,57.45 70.1,57.45 70.1,57.66 70.51,58.06 v73.97,58.06
  Bottom 0.305: v55.68,57.45 v53.24,57.45 | v73.97,58.06 73.98,58.06
  Bottom 0.406: Q6.1 78.74,69.39 78.74,72.64 73.98,72.64 73.98,58.06 73.98,57.4
D12*  (via drill 0.3)
  Top 0.305: v43.69,20.07 53.03,20.07 v53.03,31.24 | v55.47,31.45 53.03,33.88 53.03,36.32 U$4.26
  Bottom 0.305: v43.69,20.07 34.14,20.07 Q8.1 | v53.03,31.24 53.24,31.45 v55.47,31.45
D13*  (via drill 0.3)
  Top 0.305: v18.29,10.11 13.41,10.11 13.41,9.7 13.21,9.5 9.96,9.5 9.96,23.11 15.44,28.6 15.44,45.87 16.46,46.89 v16.46,52.58 | v34.14,54.61 39.83,54.61 v39.83,49.12 | v56.29,45.06 56.29,38.56 57.71,37.13 57.71,36.52 U$4.32
  Bottom 0.305: v18.29,10.11 19.51,10.11 Q9.1 | v16.46,52.58 18.49,54.61 v34.14,54.61 | v39.83,49.12 40.44,48.51 52.43,48.51 53.65,47.29 54.86,47.29 56.29,45.87 v56.29,45.06
D+USB  (via drill 0.3)
  Top 0.305: v31.29,49.73 32.72,49.73 R24.2 | v10.16,49.73 8.13,49.73 X4.3
  Bottom 0.305: v10.16,49.73 v31.29,49.73
D-USB  (via drill 0.3)
  Top 0.305: v31.5,51.16 31.5,51.56 32.72,52.78 R31.2 | v11.18,50.95 9.96,50.95 9.75,50.75 8.13,50.75 X4.2
  Bottom 0.305: v31.5,51.16 31.29,50.95 v11.18,50.95
FMOSI
  Bottom 0.305: 41.25,46.08 43.89,46.08 44.5,46.68 50.6,46.68 U$1.SI | 41.25,46.08 22.96,46.08 22.96,40.39 24.99,38.35 D5.A | 41.25,46.08 44.5,42.82 62.59,42.82 63.2,42.21 R1.1
GND  (via drill 0.3)
  Top 0.457: R2.2 69.7,52.58 v69.7,37.34 69.7,36.12 C9.2 | C11.2 66.04,43.23 66.04,40.59 R3.1 66.24,40.59 67.46,39.37 v67.46,38.56 | v62.99,36.52 62.18,37.34 62.18,38.96 60.55,38.96 U$4.35 | v77.22,38.35 77.22,45.87 U1.13 | 32.92,42.42 32.92,44.65 C2.1 32.92,44.86 v32.92,48.31 | 32.92,42.42 32.92,39.78 C8.1 | v33.12,42.42 32.92,42.42 | v49.78,52.78 49.78,53.59 51.82,53.59 C3.1 | USB.2 17.88,52.17 17.88,47.29 SERIAL.2 17.68,47.09 16.46,45.87 16.46,33.48 LED4.K 16.46,33.27 16.46,28.4 LED10.K 16.46,28.19 15.85,27.58 15.85,18.24 15.65,18.03 LED3.C | v54.66,44.25 54.66,45.47 | 54.66,45.47 54.66,45.87 55.27,46.48 55.27,47.9 U$4.5 | v57.91,45.47 60.35,45.47 U$4.43 | 50.6,43.64 48.97,43.64 U$4.15 | 50.6,43.64 50.6,36.52 U$4.23 50.6,36.32 v50.6,31.24 | v53.44,45.47 54.46,45.47 54.66,45.47 | v51.21,45.47 50.6,44.86 50.6,43.84 50.6,43.64 | IC1.1 12.19,10.72 IC1.1 | IC1.1 12.39,10.72 17.88,10.72 18.09,10.92 19.1,10.92 19.1,2.39 19.1,1.52 | X4.5 8.13,48.11 10.16,48.11 10.16,36.32 7.92,34.09 U$6.GND2 | U$3.GND 95.1,28.6 92.66,26.16 92.66,24.94 93.27,24.33 105.87,24.33 106.68,24.33
  Top 1.778: 24.13,11.68 22.54,11.68 22.54,1.52 19.1,1.52 1.27,1.52 1.27,19.3 7.62,19.3 7.62,28.15 U$6.GND1 U$6.GND2 | 24.13,11.68 45.72,11.68 | 45.72,11.68 46.99,11.68 | 46.99,11.68 62.23,11.68 | 62.23,11.68 63.5,11.68 | 63.5,11.68 78.74,11.68 | 78.74,11.68 80.01,11.68 | 80.01,11.68 95.25,11.68 | 95.25,11.68 97.79,11.68 | 97.79,11.68 106.68,11.68 106.68,24.33 106.68,73.91 100.33,73.91 | 100.33,73.91 99.06,73.91 | 99.06,73.91 85.09,73.91 | 85.09,73.91 81.28,73.91 | 81.28,73.91 68.58,73.91 | 68.58,73.91 65.28,73.91 64.77,73.91 | 64.77,73.91 51.56,73.91 50.8,73.91 | 50.8,73.91 48.77,73.91 48.26,73.91 | 48.26,73.91 35.56,73.91 | 35.56,73.91 35.05,73.91 31.75,73.91 | 31.75,73.91 18.54,73.91 17.78,73.91 | 17.78,73.91 15.88,73.91 J1.GND2 | J1.GND1 18.41,74.55 17.78,73.91 | J2.GND2 32.38,74.55 31.75,73.91 | J2.GND1 34.92,74.55 35.56,73.91 | J3.GND2 48.9,74.55 48.26,73.91 | J3.GND1 51.44,74.55 50.8,73.91 | J4.GND2 65.41,74.55 64.77,73.91 | J4.GND1 67.94,74.55 68.58,73.91 | J5.GND2 81.92,74.55 81.28,73.91 | J5.GND1 84.45,74.55 85.09,73.91 | J6.GND2 98.42,74.55 99.06,73.91 | J6.GND1 100.97,74.55 100.33,73.91 | RGB-J1.GND1 24.77,11.05 24.13,11.68 | I2C-J1.GND1 45.09,11.05 45.72,11.68 | I2C-J1.GND2 47.62,11.05 46.99,11.68 | I2C-J2.GND1 61.59,11.05 62.23,11.68 | I2C-J2.GND2 64.14,11.05 63.5,11.68 | I2C-J3.GND1 78.11,11.05 78.74,11.68 | I2C-J3.GND2 80.64,11.05 80.01,11.68 | I2C-J4.GND1 94.61,11.05 95.25,11.68 | I2C-J4.GND2 97.16,11.05 97.79,11.68
  Bottom 0.457: 91.44,27.38 93.88,27.38 95.1,28.6 U$3.GND | 91.44,27.38 87.17,27.38 86.56,27.99 85.75,27.99 85.14,28.6 U$3.SGND | 67.46,36.52 69.9,36.52 70.21,36.83 | 67.46,36.52 v62.99,36.52 | 70.21,36.83 71.32,37.95 RESET1.4 71.53,38.15 77.22,38.15 | 77.22,38.15 82.09,38.15 83.31,36.93 CFG.1 83.72,36.73 91.44,36.73 91.44,27.58 91.44,27.38 | v77.22,38.35 77.22,38.15 | v67.46,38.56 67.46,36.73 67.46,36.52 | v69.7,37.34 70.1,36.93 70.21,36.83 | C10.2 31.9,42.42 v33.12,42.42 35.56,42.42 C12.1 | 32.92,48.92 19.51,48.92 17.88,47.29 SERIAL.2 | 32.92,48.92 33.53,48.92 34.14,49.53 C7.1 34.34,49.73 37.39,52.78 v49.78,52.78 | v32.92,48.31 32.92,48.72 32.92,48.92 | RGB_5-6-11.GND 27.84,30.43 26.82,29.41 17.88,29.41 16.66,28.19 LED10.K 16.66,27.99 16.66,23.32 19.91,23.32 20.32,23.11 | v54.66,44.25 54.86,44.04 56.29,44.04 57.81,45.57 | 57.81,45.57 58.73,46.48 U$1.VSS | v57.91,45.47 57.81,45.57 | v51.21,45.47 v53.44,45.47 | 47.85,28.5 48.77,27.58 U$2.10 | 47.85,28.5 46.43,29.92 | 46.43,29.92 45.52,30.84 42.67,30.84 CON1.GND | U$2.10 48.97,27.38 U$2.10 | C1.2 6.3,12.95 6.3,15.39 C5.2 6.5,15.39 7.92,16.82 16.66,16.82 17.14,16.82 | 46.43,29.92 46.33,29.82 39.62,23.11 30.07,23.11 29.44,23.11 | v50.6,31.24 47.95,28.6 47.85,28.5
  Bottom 1.27: Q2.3 34.29,69.39 34.29,73.91 34.92,73.91 J2.GND1 | Q4.3 50.8,69.39 50.8,73.91 51.44,73.91 J3.GND1 | Q5.3 67.31,69.39 67.31,73.91 67.94,73.91 J4.GND1 | Q6.3 83.82,69.39 83.82,73.91 84.45,73.91 J5.GND1 | Q3.3 100.33,69.39 100.33,73.91 100.97,73.91 J6.GND1 | Q1.3 17.78,69.39 17.78,73.91 18.41,73.91 J1.GND1 | Q8.3 29.44,23.11 20.32,23.11 20.32,20.02 Q10.3 20.16,19.62 17.14,19.62 17.14,16.82 17.14,12.95 | Q9.3 17.23,5.56 17.14,5.65 17.14,12.95 | RGB-J1.GND1 24.77,12.64 17.46,12.64 17.14,12.95
GND1
  Bottom 0.457: LED9.C 92.86,47.09 92.86,50.95 U$3.RNU
GND2
  Bottom 0.457: LED11.C 90.22,47.09 90.22,50.95 U$3.NET
GND3
  Bottom 0.457: LED12.C 87.78,47.09 87.78,50.95 U$3.ALM
HWB  (via drill 0.3)
  Top 0.305: v59.94,32.05 59.94,35.1 58.73,36.32 U$4.33 | v61.16,32.05 64.82,35.71 64.82,37.34 66.04,38.56 R3.2
  Bottom 0.305: v61.16,32.05 v59.94,32.05
ISP+5V  (via drill 0.3)
  Top 0.305: v40.03,30.23 v42.88,27.38 | v35.76,33.27 31.29,37.74 v31.29,43.64
  Bottom 0.305: v42.88,27.38 42.67,27.38 42.67,28.19 CON1.5V | v40.03,30.23 37.59,32.66 36.37,32.66 v35.76,33.27 | v31.29,43.64 30.48,44.45 26.21,44.45 25.2,43.43 D2.A
MISO  (via drill 0.3)
  Top 0.305: v38.2,28.8 37.39,29.62 37.39,34.9 40.44,37.95 41.45,37.95 v41.45,38.35 | v44.7,41.6 45.52,42.42 v45.52,50.34 | v50.6,51.56 50.6,48.11 U$4.11
  Bottom 0.305: v38.2,28.8 40.64,28.8 41.25,28.19 CON1.MISO | v44.7,41.6 v41.45,38.35 | v45.52,50.34 46.74,51.56 v50.6,51.56 51.82,51.56 54.05,49.33 58.73,49.33 U$1.SO
MOSI  (via drill 0.3)
  Top 0.305: v44.91,35.92 v44.91,30.02 | v51.21,52.17 51.21,48.31 51.41,48.11 U$4.10 | v32.11,46.68 29.67,44.25 v29.67,39.78
  Bottom 0.305: v44.91,30.02 43.08,30.02 42.67,29.62 CON1.MOSI | v44.91,35.92 43.69,37.13 29.26,37.13 28.04,38.35 D5.C 28.25,38.35 v29.67,39.78 | v51.21,52.17 39.01,52.17 33.53,46.68 v32.11,46.68
N$1
  Bottom 0.406: Q4.2 48.26,66.29 44.45,66.29 44.45,58.67 LED6.K
  Bottom 1.27: Q4.2 48.26,73.91 46.35,73.91 J3.PWM
N$2
  Bottom 0.406: J2.I/O 31.11,80.9 40.01,80.9 R32.2
N$3
  Bottom 0.406: J6.I/O 97.16,80.9 106.68,80.9 106.68,62.48 | 106.68,62.48 106.68,56.13 | 106.68,56.13 106.68,55.18 | 106.68,55.18 106.68,56.13 | 106.68,56.13 106.68,62.48 | 106.68,55.18 106.68,56.13 | 106.68,56.13 106.68,62.48 | R19.2 106.68,54.86 106.68,56.13
N$4
  Bottom 0.406: LED5.A 35.56,58.67 R4.1
N$5
  Bottom 0.406: LED7.K 60.96,58.67 60.96,66.29 64.77,66.29 Q5.2
  Bottom 1.27: Q5.2 64.77,73.91 62.87,73.91 J4.PWM
N$6  (via drill 0.3)
  Top 0.305: v27.43,18.64 27.43,19.46 29.06,21.08 29.06,29.41 33.33,29.41 RL9.1
  Bottom 0.305: v27.43,18.64 27.3,18.03
  Bottom 1.27: RGB-J1.G 27.3,18.03 22.86,18.03 Q10.2
N$7
  Bottom 0.406: J3.I/O 47.62,80.9 56.52,80.9 R33.2
N$8
  Bottom 0.305: RL1.2 23.16,52.38 20.32,52.38 USB.3
N$9
  Bottom 0.406: LED1.A 101.6,58.67 R20.1
N$10
  Bottom 0.305: R17.1 62.38,48.51 62.38,50.95 62.18,50.95 R16.1 61.98,50.95 59.33,50.95 58.93,50.55 U$1.CE
N$11
  Bottom 0.305: R11.2 90.22,32.26 90.22,28.8 U$3.RX1
N$12
  Top 0.305: RL4.2 21.54,34.09 19.1,34.09 19.1,33.27 LED4.A
N$13
  Bottom 0.305: RL5.2 23.16,47.29 20.32,47.29 SERIAL.3
N$14
  Bottom 0.305: RL7.2 12.39,52.38 15.24,52.38 USB.1
N$15
  Bottom 0.305: RL6.2 12.39,47.29 15.24,47.29 SERIAL.1
N$16
  Top 0.305: U$4.6 54.66,48.11 54.66,53.59 C3.2
N$17
  Bottom 0.406: LED2.A 19.05,58.67 R25.1
N$18
  Bottom 0.406: J1.I/O 14.61,80.9 23.5,80.9 R.2
N$19
  Bottom 0.406: Q6.2 81.28,66.29 77.47,66.29 77.47,58.67 LED8.K
  Bottom 1.27: Q6.2 81.28,73.91 79.38,73.91 J5.PWM
N$20
  Top 0.305: LED3.A 17.48,18.03 17.48,15.6 R27.1
N$21
  Bottom 0.406: Q3.2 97.79,66.29 93.98,66.29 93.98,58.67 LED1.K
  Bottom 1.27: Q3.2 97.79,73.91 95.89,73.91 J6.PWM
N$22
  Bottom 0.406: LED6.A 52.07,58.67 R5.1
N$23  (via drill 0.3)
  Top 0.305: v67.46,46.89 v67.46,45.67 | v62.59,46.89 55.88,46.89 55.88,46.08 v55.47,45.67
  Bottom 0.305: v67.46,45.67 67.06,45.67 66.24,44.86 R18.2 | v62.59,46.89 v67.46,46.89 | v55.47,45.67 54.46,46.68 52.63,46.68 51.61,47.7 50.8,47.7 U$1.SCK
N$24
  Bottom 0.305: R8.2 87.58,32.26 87.58,28.8 U$3.TX1
N$25
  Bottom 0.305: LED9.A 92.86,44.86 92.86,42.01 R12.1
N$26
  Bottom 0.305: LED11.A 90.22,44.86 90.22,42.01 R14.1
N$27
  Bottom 0.305: LED12.A 87.78,44.86 87.78,42.01 R39.1
N$28
  Bottom 0.406: Q2.2 31.75,66.29 27.94,66.29 27.94,58.67 LED5.K
  Bottom 1.27: Q2.2 31.75,73.91 29.84,73.91 J2.PWM
N$29
  Bottom 0.406: J4.I/O 64.14,80.9 73.03,80.9 R34.2
N$30
  Bottom 0.406: LED7.A 68.58,58.67 R6.1
N$32
  Bottom 0.406: J5.I/O 80.64,80.9 89.53,80.9 R35.2
N$33
  Bottom 0.406: LED8.A 85.09,58.67 R7.1
N$34
  Bottom 0.406: Q1.2 15.24,66.29 11.43,66.29 11.43,58.67 LED2.K
  Bottom 1.27: Q1.2 15.24,73.91 13.34,73.91 J1.PWM
N$35  (via drill 0.3)
  Top 0.305: v73.97,44.04 74.17,44.25 74.17,50.34 74.78,50.95 U$3.CFG
  Bottom 0.305: v73.97,44.04 77.62,44.04 79.05,42.62 CFG.4
N$36
  Top 0.305: RL2.2 35.15,32.05 34.34,32.87 34.34,33.07 34.14,33.27 28.04,33.27 28.04,32.66 RGB_5-6-11.RED
N$37  (via drill 0.3)
  Top 0.305: v29.67,27.38 29.67,26.98 33.33,26.98 RL8.2
  Bottom 0.305: v29.67,27.38 28.85,26.57 28.04,26.57 RGB_5-6-11.BLU
N$38  (via drill 1.1)
  Top 1.778: v1.27,72.64 1.27,74.5 F2.1
  Bottom 1.778: U$6.+5V 11.35,34.62 7.62,38.35 7.62,42.16 1.27,42.16 v1.27,72.64
N$39
  Bottom 1.778: U$6.+12V 11.35,26.84 7.62,23.11 7.62,19.3 1.27,19.3 1.27,2.79 5.08,2.79 F1.1
N$40  (via drill 0.3)
  Top 0.305: v34.34,28.19 34.34,28.6 35.15,29.41 RL9.2
  Bottom 0.305: v34.34,28.19 34.14,28.4 28.04,28.4 RGB_5-6-11.GRN
N$42
  Top 0.305: C8.2 35.76,39.57 39.22,39.57 X3.P$2 39.42,39.78 43.08,39.78 43.08,40.59 R13.2 43.28,40.79 44.91,40.79 45.92,41.81 45.92,42.01 48.77,42.01 U$4.17
N$50  (via drill 0.3)
  Top 0.305: v32.51,24.13 35.15,26.77 RL8.1 | v19.91,9.09 v19.91,24.13
  Bottom 0.305: v19.91,24.13 v32.51,24.13 | v19.91,9.09 19.91,8.48 19.91,7.87
  Bottom 1.27: Q9.2 19.91,7.87 22.86,7.87 22.86,4.06 28.57,4.06 RGB-J1.B
N$68  (via drill 0.3)
  Top 0.305: v32.92,20.88 36.37,24.33 36.37,30.63 34.54,30.63 34.14,31.04 34.14,31.24 33.53,31.85 RL2.1
  Bottom 0.305: v32.92,20.88 32.31,20.27 Q8.2
  Bottom 1.27: RGB-J1.R 29.84,17.72 31.75,17.72 Q8.2
N$70  (via drill 0.3)
  Top 0.305: v66.85,54.41 63.6,54.41 R10.1 | v91.24,54.2 94.08,51.36 94.08,47.7 95.1,46.68 95.1,46.08 U1.1
  Bottom 0.305: v66.85,54.41 67.06,54.2 v91.24,54.2
N$75
  Top 0.305: RL3.1 21.54,29.01 19.1,29.01 19.1,28.19 LED10.A
RD+  (via drill 0.3)
  Top 0.305: v34.34,50.95 35.56,49.73 R24.1 35.36,50.14 v39.22,54 | v56.08,51.97 56.08,48.11 U$4.4
  Bottom 0.305: v34.34,50.95 33.33,50.95 32.72,50.34 10.57,50.34 10.57,52.17 RL7.1 | v56.08,51.97 54.05,54 v39.22,54
RD-  (via drill 0.3)
  Top 0.305: v34.34,53.8 35.56,53.8 35.56,52.98 R31.1 | v56.08,52.98 56.9,52.17 56.9,48.11 U$4.3
  Bottom 0.305: RL1.1 25.2,52.38 26.62,53.8 v34.34,53.8 35.15,54.61 54.46,54.61 v56.08,52.98
RESET  (via drill 0.3)
  Top 0.305: 67.87,33.48 69.7,33.48 69.7,33.27 C9.1 | 67.87,33.48 66.04,33.48 R15.1 | v46.74,50.14 46.74,45.47 48.77,45.47 U$4.13 | v38.41,49.73 34.54,45.87 34.54,35.51 v36.78,33.27 | v67.87,32.26 67.87,33.48
  Bottom 0.305: 42.06,33.27 42.06,31.85 41.45,31.24 41.45,30.84 CON1.RESET | 42.06,33.27 63.6,33.27 64.62,32.26 v67.87,32.26 70.1,32.26 71.32,33.48 RESET1.2 | v46.74,50.14 46.33,49.73 v38.41,49.73 | 42.06,33.27 v36.78,33.27
RX  (via drill 0.3)
  Top 0.305: v48.77,32.05 48.77,35.51 47.75,36.52 47.75,39.57 48.77,39.57 U$4.20 | v63.6,31.45 71.12,31.45 v71.12,31.85 71.12,36.93 70.31,37.74 70.31,47.9 v70.51,48.11 | v66.04,52.58 63.6,52.58 R10.2
  Bottom 0.305: v48.77,32.05 48.97,31.85 52.83,31.85 53.03,32.05 58.93,32.05 59.54,31.45 v63.6,31.45 | v71.12,31.85 71.53,32.26 85.55,32.26 87.38,34.09 87.58,34.09 R8.1 | v70.51,48.11 v66.04,52.58
RXLED  (via drill 0.3)
  Top 0.305: v28.65,48.11 30.89,50.34 30.89,53.19 34.95,57.25 47.95,57.25 v47.95,55.63 | v53.03,51.36 53.03,48.11 U$4.8
  Bottom 0.305: v28.65,48.11 26.01,48.11 25.2,47.29 RL5.1 | v47.95,55.63 48.36,55.22 54.86,55.22 56.69,53.39 56.69,51.36 v53.03,51.36
SCK  (via drill 0.3)
  Top 0.305: v39.83,29.41 39.42,29.82 39.42,33.48 v45.92,39.98 | v52.02,41 52.22,41.2 v52.22,43.43 | v53.44,43.43 53.44,44.45 52.43,45.47 52.43,47.7 52.22,47.9 U$4.9
  Bottom 0.305: v39.83,29.41 41.25,29.41 CON1.SCK | v45.92,39.98 46.94,41 v52.02,41 | v52.22,43.43 v53.44,43.43 61.98,43.43 63.2,44.65 R18.1
SCL  (via drill 0.3)
  Top 0.305: v52.43,24.13 52.43,25.35 47.55,30.23 47.55,35.1 46.53,36.12 46.53,41.2 48.77,41.2 U$4.18 | v59.13,25.35 v57.3,23.52
  Bottom 0.305: v52.43,24.13 53.03,23.52 v57.3,23.52 | 58.83,25.65 57.91,26.57 57.91,27.38 U$2.3 | 58.83,25.65 v59.13,25.35 | R28.2 63.8,26.77 63.8,25.76 58.93,25.76 58.83,25.65
SCL1  (via drill 0.3)
  Top 0.305: v77.22,30.63 78.84,29.01 v78.84,24.33
  Bottom 0.305: v77.22,30.63 58.32,30.63 57.1,29.41 55.27,29.41 55.27,27.58 U$2.5 | v78.84,24.33 79.45,23.72 97.54,23.72 99.97,21.29 R30.2
  Bottom 0.406: I2C-J4.SCL 99.69,18.03 99.83,18.03 R30.2
SCL2  (via drill 0.3)
  Top 0.305: v53.65,30.63 56.69,27.58 56.69,22.71 59.94,19.46 59.94,19.25 60.15,19.05 73.36,19.05 73.36,19.25 v77.01,22.91
  Bottom 0.305: v53.65,30.63 51.61,30.63 51.61,27.58 U$2.8 | v77.01,22.91 77.42,22.5 83.52,22.5 84.73,21.29 R37.1
  Bottom 0.406: I2C-J3.SCL 83.19,18.03 84.9,18.03 R37.1
SCL3  (via drill 0.3)
  Top 0.305: v46.53,35.1 46.33,34.9 v46.33,27.99
  Bottom 0.305: v46.53,35.1 49.99,35.1 49.99,36.52 U$2.12 | v46.33,27.99 48.97,25.35 57.1,25.35 57.71,24.74 61.37,24.74 63.6,22.5 67.06,22.5 68.28,21.29 R22.1
  Bottom 0.406: I2C-J2.SCL 66.67,18.03 68.39,18.03 R22.1
SCL4  (via drill 0.3)
  Top 0.305: v45.92,38.76 44.3,37.13 v44.3,23.52
  Bottom 0.305: v45.92,38.76 53.85,38.76 53.85,36.73 U$2.15 | v44.3,23.52 45.31,22.5 50.6,22.5 51.82,21.29 R23.1
  Bottom 0.406: I2C-J1.SCL 50.16,18.03 51.88,18.03 R23.1
SDA  (via drill 0.3)
  Top 0.305: v48.16,31.45 48.16,35.31 47.14,36.32 47.14,40.39 48.77,40.39 U$4.19 | v46.94,30.43 46.94,28.4 v52.43,22.91 | v60.35,22.91 62.59,22.91 v62.59,26.37
  Bottom 0.305: v48.16,31.45 47.14,30.43 v46.94,30.43 | v60.35,22.91 v52.43,22.91 | 62.59,29.01 62.59,29.41 63.8,29.41 R29.2 | 62.59,29.01 v62.59,26.37 | 62.59,29.01 57.51,29.01 57.3,28.8 56.69,28.8 56.69,27.58 U$2.4
SDA1  (via drill 0.3)
  Top 0.305: v56.69,30.02 57.51,30.02 59.94,27.58 73.56,27.58 v77.62,23.52
  Bottom 0.305: v56.69,30.02 54.05,30.02 54.05,27.58 U$2.6 | v77.62,23.52 78.03,23.11 91.03,23.11 92.86,21.29 R36.1
  Bottom 0.406: I2C-J4.SDA 98.42,4.7 92.71,4.7 92.71,12.32 95.25,12.32 95.25,18.03 92.9,18.03 R36.1
SDA2  (via drill 0.3)
  Top 0.305: v58.12,25.35 58.73,25.96 61.98,25.96 v61.98,25.15
  Bottom 0.305: v58.12,25.35 57.51,25.96 50.19,25.96 50.19,27.38 U$2.9 | v61.98,25.15 64.01,23.11 75.79,23.11 77.62,21.29 R38.1
  Bottom 0.406: I2C-J3.SDA 81.92,4.7 76.2,4.7 76.2,12.32 78.74,12.32 78.74,18.03 77.66,18.03 R38.1
SDA3  (via drill 0.3)
  Top 0.305: v43.69,35.1 42.06,33.48 42.06,29.21 43.69,27.58 v43.69,26.16
  Bottom 0.305: v43.69,35.1 45.11,35.1 48.16,38.15 51.41,38.15 51.41,36.73 U$2.13 | v43.69,26.16 45.11,24.74 56.9,24.74 57.51,24.13 60.15,24.13 61.16,23.11 61.16,21.29 R26.1
  Bottom 0.406: I2C-J2.SDA 65.41,4.7 59.69,4.7 59.69,12.32 62.23,12.32 62.23,18.03 61.15,18.03 R26.1
SDA4  (via drill 0.3)
  Top 0.305: v73.36,43.43 74.17,42.62 74.17,31.24 76.2,29.21 76.2,25.96 78.23,23.93 78.23,23.11 73.15,18.03 v45.72,18.03
  Bottom 0.305: v73.36,43.43 65.02,43.43 65.02,41.6 64.21,40.79 59.94,40.79 59.54,40.39 54.86,40.39 54.86,38.76 55.07,38.56 55.07,36.73 U$2.16
  Bottom 0.406: I2C-J1.SDA 48.9,4.7 43.18,4.7 43.18,12.32 45.72,12.32 v45.72,18.03 44.64,18.03 R21.2
TX  (via drill 0.3)
  Top 0.305: v52.43,32.46 52.43,30.63 50.19,30.63 49.99,30.84 49.99,38.96 48.97,38.96 U$4.21 | v72.34,31.24 v72.34,35.31 72.34,52.58 R9.2
  Bottom 0.305: v52.43,32.46 52.63,32.66 63.4,32.66 64.82,31.24 v72.34,31.24 | v72.34,35.31 89,35.31 90.02,34.29 R11.1
TXLED  (via drill 0.3)
  Top 0.305: v38,34.49 38.81,33.68 38.81,27.99 43.89,22.91 45.72,22.91 v45.72,31.65 | v49.38,32.66 49.38,37.74 48.97,38.15 U$4.22
  Bottom 0.305: v38,34.49 23.16,34.49 10.57,47.09 RL6.1 | v45.72,31.65 46.74,32.66 v49.38,32.66
VUSB  (via drill 0.3)
  Top 0.305: v53.65,51.97 53.65,48.11 U$4.7 | v14.83,46.08 11.79,49.12 11.79,51.36 11.68,51.46 | 11.68,51.46 11.58,51.56 8.13,51.56 X4.1 | v28.04,53.19 26.21,55.02 26.21,56.84 25.2,57.86 17.07,57.86 17.07,56.84 11.79,51.56 11.68,51.46
  Bottom 0.305: v53.65,51.97 52.22,53.39 35.15,53.39 34.34,52.58 C7.2 34.14,52.58 33.53,53.19 v28.04,53.19 | v14.83,46.08 23.57,37.34 26.62,37.34 26.62,39.37 25.2,40.79 D4.A
XTAL1  (via drill 0.3)
  Top 0.305: v46.13,43.43 46.13,43.03 48.77,43.03 U$4.16 | v44.91,43.43 43.28,43.43 R13.1 43.08,43.64 39.42,43.64 39.42,44.65 X3.P$1 39.22,44.65 35.76,44.65 C2.2
  Bottom 0.305: v44.91,43.43 v46.13,43.43

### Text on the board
tNames: BioReactor | Control Board v2 | 1 | 1 | w5100
bNames: USB | TX/RX | LINKLED
203bmp: C:/Users/G/Pictures/logo_epfl.bmp

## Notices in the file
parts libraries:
lpatiny: ©2009 ROFA.cz - modified and updated by Robert Darlington ‹rdarlington@gmail.com›
SparkFun: Licensing: CC v3.0 Share-Alike You are welcome to use this library for commercial purposes.
